FUNCTION "abvspu_AMP" : VOID
TITLE = Analoge Messwertverarbeitung
//
// Analoge Messwertverarbeitung
//
// History:
// --------
// 26-Aug-2005
// - Fehler bei cancel <out of range>
// 06-Nov-2004
// - Struktur DB180/181 erweitert (UndefGrp)
// 04-Feb-2004 (fixed)
// - TITLE = Messwert bilden (TYPE=1,...,15) - Eingangs-MS
//   U     DBX [AR1,P#21.7]; //unquittiert
//   // diese Abfrage entfernt! Relikt aus nicht optimierter SPU
//   U     #bUndefined;
//   SPB   M016;
//
// 16-Mai-2003 (added)
// - TITLE = Messwertänderung
//   Messwert-Kompensation
// - TITLE = Dyn. Limits
//   Refaktorisiert
//
// 05-Feb-2003 (redesign: Optimierung auf Geschwindigkeit)
//
AUTHOR : ab_rfe
FAMILY : AbvSpu
NAME : ANA_MS
VERSION : 3.2


VAR_INPUT
  OBJ : INT ;	// OBJ
  _TYPE : INT ;	// TYPE
  IN_VALUE : DWORD ;	// Analoger Eingangswert
  MSD_DBNO : WORD ;	// MS-Datenfeld (DB-Nummer)
  MSD_OFFSET : WORD ;	// MS-Datenfeld (Byteoffset)
  UNDEF_GRP : WORD ;	// Undefined Group
END_VAR
VAR_OUTPUT
  OUT_VALUE : WORD ;	// Ausgangswert (PAW)
  OUT_FLAG : BOOL ;	// Flag (new out_value)
END_VAR
VAR_TEMP
  help_db1 : WORD ;
  dwadr_db2_limits : WORD ;	// Anfang <Limits> in HilfsDB2
  r4NormVal : REAL ;	// aktueller Messwert (normiert)
  r4RawVal : REAL ;	// aktueller Messwert (Rohwert)
  bUndefined : BOOL ;
  bOutOfRange : BOOL ;
  bFadedOut : BOOL ;
  bAOValChanged : BOOL ;
  wRawVal : WORD ;	// Rohwert (gefiltert)
  wRawVal0 : WORD ;	// Rohwert (ungefiltert)
  dRawVal : DWORD ;
  yAnzStates : BYTE ;
  ySklRefNo : BYTE ;
  wParaDB : WORD ;	//DB-Nr. MS-Parameter
  dXmpStart : DWORD ;	// Zeiger auf Anfang MS-Datenfeld
  dXmpStates : DWORD ;	// Zeiger auf Zustandsdatenfeld
  dXmpAnaVars : DWORD ;	// Zeiger auf Zustandsdatenfeld
  dXmpLimits : DWORD ;	// Zeiger auf Zustandsdatenfeld
  dXmpLimitsEnd : DWORD ;	// Zeiger auf Zustandsdatenfeld
  dAR_UndefGrps : DWORD ;	// ptr -> Byte-Array UndefGrps
  dAR1 : DWORD ;
  dAR2 : DWORD ;
  wTmp : WORD ;
  wCycle1Ms : WORD ;
  bGA_Required : BOOL ;	// GA-Anforderung von DB104.DBX171.0
  yNewStatus : BYTE ;	//neuer Zustand
  yMB232 : BYTE ;
  yMB233 : BYTE ;
  r4LmtTemp : REAL ;
  r4LmtSaved : REAL ;
  r4LmtHysteresis : REAL ;
  wNewLvl : WORD ;
  wCurrDelay : WORD ;
  bValueAscending : BOOL ;	// Messwert steigend
  bValueDecreasing : BOOL ;	// Messwert fallend
  bLmtSaved : BOOL ;	// gerettetes Limit vorhanden
  bCheckOutOfRange : BOOL ;	// <OutOfRange> pruefen
  iObjKMS : INT ;	// Objektnummer Kompensations-MS
  r4ValKMS : REAL ;	// Messwert Kompensations-MS
  bRetValKMS : BOOL ;
  bLmtChanged : ARRAY  [1 .. 7 ] OF BOOL ;
  bLmtLast : BOOL ;
  wAnzLmts : INT ;
  r4MBA : REAL ;
  r4MBE : REAL ;
END_VAR
BEGIN
NETWORK
TITLE = Initialisierung

      L     "abvspu_DB_GLO".Cycle1Ms; // Zykluszeit (1ms-Aufl”sung)
      T     #wCycle1Ms;

      CLR   ;
      =     #bUndefined;

      L     #UNDEF_GRP;
      L     0;
      ==D   ;
      SPB   a001;

      L     "abvspu_DB_GLO".AR_UndefGrps;
      T     #dAR_UndefGrps;

      AUF   "abvspu_DB_GLO";
      LAR1  #dAR_UndefGrps;
      L     #UNDEF_GRP;
      +     -1;
      L     1; // 1 byte pro UndefGrp
      *D    ;
      SLD   3;
      +AR1  ;
      L     DBB [AR1,P#0.0];
      L     0;
      <>D   ;
      =     #bUndefined;

a001: NOP   0;
      L     #MSD_DBNO;
      T     #wParaDB;
      L     #MSD_OFFSET;
      SLD   3;
      T     #dXmpStart;
      LAR1  ;
      +AR1  P#26.0; //+13dw
      TAR1  #dXmpStates;

      CLR   ;
      =     #bOutOfRange;

      =     #bFadedOut;
      =     #bLmtSaved;

      =     #bValueAscending;
      =     #bValueDecreasing; // Nr. HilfsDB1 merken

      L     0; // HilfsDB1 aufrufen
      T     #yNewStatus; // Generalabfrage
      L     "spuDB_CFG".D_52; // DB195.DBW104
      T     #help_db1;

      AUF   DB [#help_db1];
      U     DBX  171.0;
      =     #bGA_Required;
NETWORK
TITLE = Feldbereiche berechnen

      AUF   DB [#wParaDB]; // Parameter-DB oeffnen
      LAR1  #dXmpStart;

      L     DBB [AR1,P#0.0]; // Kennung Ana-MS
      L     W#16#2; // Typ = ANA
      ==I   ;
      SPB   M001;
      L     W#16#B302; // falscher Feldtyp
      BEA   ;
M001: NOP   0;

      L     DBB [AR1,P#1.0]; // Anzahl Zustaende
      T     #yAnzStates;

      INC   1; // Zustand <OutOfRange>
      L     12; // 6DWs pro Zustand
      *I    ;
      SLD   3;
      L     #dXmpStates;
      +D    ;
      T     #dXmpAnaVars;
      L     34; //+17dw
      SLD   3;
      +D    ;
      T     #dXmpLimits;

      L     #yAnzStates;
      DEC   1;
      L     14; // Limitfeld (7dw)
      *I    ;
      SLD   3;
      L     #dXmpLimits;
      +D    ;
      T     #dXmpLimitsEnd; // ptr -> Ende Limitfeld

NETWORK
TITLE = Generalabfrage

      U     #bGA_Required; // Generalabfrage
      S     DBX [AR1,P#3.1]; // GA-Bit 'Zustand/Messwert'
      S     DBX [AR1,P#3.3]; // GA-Bit 'Nachparametrierung'
NETWORK
TITLE =Zeitverzögerung (current delay)

      UN    DBX [AR1,P#20.4]; // delay gestartet
      SPB   M002;
      L     DBW [AR1,P#22.0];
      L     #wCycle1Ms; // Zykluszeit (1ms-Auflösung)
      -I    ;
      T     DBW [AR1,P#22.0];
      L     0; // Stufe 1 abgearbeitet
      >I    ;
      SPB   M002;
      L     DBW [AR1,P#12.0]; // Zeitstufe 2
      +     -1;
      T     DBW [AR1,P#12.0];

      L     DBW [AR1,P#22.0];
      +     1000;
      T     DBW [AR1,P#22.0]; // Stufe 1 neu laden

M002: NOP   0;
NETWORK
TITLE = scancycle



NETWORK
TITLE =Grenzwerthysterese

      LAR2  #dXmpAnaVars; // ptr -> Analogvariablen
      L     DBD [AR2,P#8.0]; // Grenzwerthysterese/2
      T     #r4LmtHysteresis;

NETWORK
TITLE = Messwert bilden (TYPE=256) - Ausgangs-MS

      L     #_TYPE;
      L     256;
      <I    ;
      SPB   M003; // Eingangs-MS

      CLR   ;
      =     #OUT_FLAG;

      L     DBD [AR1,P#16.0]; // Messwert via SetValue()
      T     #r4NormVal;

      U     DBX [AR1,P#3.1]; // GA-Bit 'Zustand/Messwert'
      O(    ;
      L     #r4NormVal; // neuer Messwert
      L     DBD [AR1,P#4.0]; // aktueller Messwert
      <>R   ;
      )     ;
      =     #bAOValChanged;
      U     #bAOValChanged;
      SPB   M004;
      L     DBW [AR1,P#14.0];
      SPA   M005;
M004: NOP   0;
// Messwertaenderung=>Ausgang ansteuern;
// Messwert normieren (invers);
      L     1.000000e+000;
      L     DBD [AR2,P#0.0]; // a-Wert
      /R    ;
      L     #r4NormVal;
      *R    ;
      L     DBD [AR2,P#4.0]; // b-Wert
      +R    ;
      TRUNC ;
      T     #wRawVal;
      T     DBW [AR1,P#14.0];
      NOP   0;
//check range
M005: L     DBW [AR2,P#20.0]; //UNGR
      ITD   ;
      <D    ;
      SPB   M006;
      TAK   ;
      L     DBW [AR2,P#22.0]; //OBGR
      ITD   ;
      <=D   ;
      SPB   M007;
M006: NOP   0;
//OutOfRange
      L     16;
      T     #yNewStatus;
      SPA   M008;
M007: NOP   0;
// Rohwert ausgeben
      UN    #bAOValChanged;
      SPB   M008;
      CLR   ;
      L     #wRawVal;
      T     #OUT_VALUE;
      SET   ;
      =     #OUT_FLAG;
      SPA   M008;
NETWORK
TITLE = Messwert bilden (TYPE=1,...,15) - Eingangs-MS

M003: NOP   0;
      L     #_TYPE;
      L     15;
      >I    ; // wenn Type > 15 dann physikal.
      SPB   M009;

      NOP   0;
//Hardware-Signal einlesen;
      L     #IN_VALUE;
      T     #wRawVal;
      T     #wRawVal0;

      L     #_TYPE;
      SPL   M010;
      SPA   M011;
      SPA   M012; // HWM=1
      SPA   M011; // HWM=2 (PT100)
M010: NOP   0;
M011: NOP   0;
//Rohwert uebernehmen
      L     #wRawVal0;
      T     #wRawVal;
      SPA   M013;
M012: NOP   0;
//Rohwert maskieren
      L     #wRawVal0;
      UW    W#16#FFF8;
      T     #wRawVal;
      SPA   M013;
M013: NOP   0;
//bit 0,1,2 pruefen;
//bit 0: Ueberlauf;
//bit 1: Fehler
//bit 2: ?
//Undefined-Erkennung via UndefGrp
      U     #bUndefined;
      SPB   M014;
//Undefined-Erkennung via Rohwert
      L     #wRawVal0;
      L     W#16#7FFF;
      ==I   ;
      SPB   M014;
      TAK   ;
      L     W#16#8000;
      ==I   ;
      SPB   M014;
      SPA   M015;
M014: NOP   0;
      L     17; // undefiniert in UebergabeDW
      T     #yNewStatus;
M015: NOP   0;
      L     #wRawVal0;
      L     W#16#FFFE; // letztes Messwertbit ausblenden
      UW    ;
      T     #wRawVal; // aktueller Rohwert
      L     DBW [AR2,P#26.0]; // alter Rohwert
      ==I   ;
      =     DBX [AR1,P#20.2]; // Messwert gleich
      TAK   ;
      T     DBW [AR2,P#26.0]; // Messwert uebernehmen

      U     #bUndefined;
      SPB   M016;
      L     DBW [AR2,P#26.0]; // aktueller Messwert
      L     DBW [AR2,P#20.0]; // UNGR for out of range
      <I    ;
      SPB   M017;
      TAK   ;
      L     DBW [AR2,P#22.0]; // OBGR for out of range
      <=I   ;
      SPB   M016;
M017: NOP   0;
//OutOfRange
      L     16;
      T     #yNewStatus;
M016: NOP   0;
//normierten Messwert bilden;
      L     #wRawVal;
//konvertiere INT_16 nach INT_32;
//Wird Vorzeichen beruecksichtigt?
      ITD   ;
      T     #dRawVal;
//konvertiere INT_32 nach Real
      DTR   ;
      T     #r4RawVal;
      U     #bUndefined; // Messwert undefiniert
      SPB   M018;
      L     DBB [AR2,P#24.0]; // SKL-RefNo (wenn > 0 dann Normierung mit Polygon)
      T     #ySklRefNo;
      L     0;
      <>I   ;
      SPB   M019;
// Messwert normieren;
      L     DBD [AR2,P#0.0]; // a-Wert
      L     #r4RawVal; // x-Wert (Rohwert als Real)
      *R    ;
      L     DBD [AR2,P#4.0]; // b-Wert
      +R    ;
      T     #r4NormVal; // normierter Messwert
      SPA   M008; // ->Messwertvergleich
M019: NOP   0;
// normierter Messwert
      CALL "abvspu_XPO_NORM" (
           PODX                     := #ySklRefNo,
           ROHW                     := #r4RawVal,
           NRMV                     := #r4NormVal);

      SPA   M008;
M018: NOP   0;
      L     1.000000e+006;
      T     #r4NormVal; // normierter Messwert
      SPA   M008;
NETWORK
TITLE = Messwert bilden (physikalisch)

M009: NOP   0;
      L     #_TYPE;
      L     16; // physikal. Messwert 16 BIT
      ==I   ;
      SPB   M020;
// *** 32 BIT Wert ***;
      L     0.000000e+000;
      L     #IN_VALUE;
      +R    ;
      UN    UO; // Gleitpunktzahl gueltig
      SPB   REOK;
      L     #r4NormVal; // alten phys. Messwert beibehalten
REOK: T     #r4NormVal; // phys. Messwert (real)
      SPA   M021;
M020: NOP   0;
// *** 16 BIT Wert ***;
      L     #IN_VALUE;
      T     #wRawVal; // phys. Messwert (int16)
      ITD   ;
      T     #dRawVal;
      DTR   ; // ->real
      T     #r4NormVal; // Wert als Real
//*** Start: OutOfRange (pysikalisch) ***//
M021: NOP   0;

      L     DBB [AR2,P#24.0]; // SKL-RefNo (wenn > 0 dann Normierung mit Polygon)
      T     #ySklRefNo;
      L     0;
      ==I   ;
      SPB   M022;
// normierter Messwert
      CALL "abvspu_XPO_NORM" (
           PODX                     := #ySklRefNo,
           ROHW                     := #r4NormVal,
           NRMV                     := #r4NormVal);

      AUF   DB [#wParaDB];
      LAR1  #dXmpStart;
      LAR2  #dXmpAnaVars;

M022: NOP   0;
      L     #r4NormVal;
      L     DBD [AR2,P#0.0]; //Messbereichsanfang
      <R    ;
      SPB   M023;
      TAK   ;
      L     DBD [AR2,P#4.0]; //Messbereichsende
      <=R   ;
      SPB   M024;
M023: NOP   0;
//OutOfRange
      L     16;
      T     #yNewStatus;
      SPA   M027;
M024: NOP   0;
      UN    #bUndefined;
      SPB   M027;
      L     17; // undefiniert in UebergabeDW
      T     #yNewStatus;
M027: NOP   0;
//*** Ende : OutOfRange (pysikalisch) ***//
NETWORK
TITLE = Messwertaenderung?

M008: NOP   0;

      LAR2  #dXmpAnaVars;
      L     DBW [AR2,P#28.0]; // ObjNo Kompensations-MS
      L     0;
      ==I   ;
      SPB   wei3;
//
// Kompensations-MS
      TAK   ;
      T     #iObjKMS;

      CALL "GetValueR_ex" (
           obj                      := #iObjKMS,
           rVal                     := #r4ValKMS,
           bOk                      := #bRetValKMS);

      UN    #bRetValKMS;
      SPB   wei3;

// cancel <out of range>
//    L     0;
//    T     #yNewStatus;

      L     #r4NormVal;
      L     #r4ValKMS;
      +R    ;
      T     #r4NormVal;
      SPA   wei3;

// raw value zurückrechnen, um 'out of range' zu prüfen
      L     1.000000e+000;
      L     DBD [AR2,P#0.0]; // a-Wert
      /R    ;
      L     #r4NormVal;
      *R    ;
      L     DBD [AR2,P#4.0]; // b-Wert
      +R    ;
      TRUNC ; // raw value

//check range
      L     DBW [AR2,P#20.0]; //UNGR
      ITD   ;
      <D    ;
      SPB   k001;
      TAK   ;
      L     DBW [AR2,P#22.0]; //OBGR
      ITD   ;
      <=D   ;
      SPB   wei3;
k001: NOP   0;
//OutOfRange
      L     16;
      T     #yNewStatus;

wei3: NOP   0;
      UN    DBX [AR1,P#3.2]; // Simulationsmodus?
      SPB   M025;
      L     #OBJ; // ObjNo
      T     #wTmp;
      L     #r4NormVal; // Akt. Messwert -> Akku1
      CALL "abvspu_AMPSIM" (
           OBJ                      := #wTmp);

      T     #r4NormVal; // Aktueller Messwert
M025: NOP   0;
      L     #r4NormVal;
      L     DBD [AR1,P#4.0]; //alter Messwert
      ==R   ;
      =     DBX [AR1,P#20.2]; // Messwert gleich

// force value changed, if <status==0> or <GA-Bit>
      L     DBW [AR1,P#8.0];
      L     0;
      ==I   ;
      O     DBX [AR1,P#3.1];
      O     DBX [AR1,P#3.4]; // force value change
      R     DBX [AR1,P#20.2]; // Messwert gleich

      UN    DBX [AR1,P#20.2];
      =     DBX [AR1,P#20.7]; // Messwert eintragen

      U     DBX [AR1,P#3.4];
      R     DBX [AR1,P#3.4];
NETWORK
TITLE = Dynamische Limits

      L     0;
      L     DBB [AR2,P#33.0];
      ==I   ; // dynamische Limits vorhanden?
      SPB   M026;

      CLR   ;
      =     #bLmtChanged[1];
      =     #bLmtChanged[2];
      =     #bLmtChanged[3];
      =     #bLmtChanged[4];
      =     #bLmtChanged[5];
      =     #bLmtChanged[6];
      =     #bLmtChanged[7];

//Messbereichsanfang, -ende ermitteln
      L     #_TYPE;
      L     16;
      >=I   ;
      O(    ;
      L     #ySklRefNo; // Skaliergruppe
      L     0;
      >I    ;
      )     ;
      SPB   RNG2;
//Messbereich aus Gradient/Offset ermitteln;
//MBA=offset+(gradient*UNGR)
//MBE=(gradient*OBGR)+offset
      L     DBW [AR2,P#20.0]; //UNGR
      ITD   ;
      DTR   ;
      L     DBD [AR2,P#0.0]; //Gradient
      *R    ;
      L     DBD [AR2,P#4.0]; //Offset
      +R    ;
      T     #r4MBA;
//
      L     DBW [AR2,P#22.0]; //OBGR
      ITD   ;
      DTR   ;
      L     DBD [AR2,P#0.0]; //Gradient
      *R    ;
      L     DBD [AR2,P#4.0]; //Offset
      +R    ;
      T     #r4MBE;
      SPA   RNGX;
RNG2: NOP   0;
      L     DBD [AR2,P#0.0];
      T     #r4MBA;
      L     DBD [AR2,P#4.0];
      T     #r4MBE;

RNGX: NOP   0;

      L     #yAnzStates; // Anzahl Zustaende
      +     -1; // Anzahl Limits
      T     #wAnzLmts;

      UN    DBX [AR2,P#33.1]; // 1. Limit dynamisch
      SPB   LIM2;


      CALL "abvspu_DYLI" (
           IN_Obj                   := #OBJ,
           IN_wParaDB               := #wParaDB,
           IN_dXmpAnaVars           := #dXmpAnaVars,
           IN_dXmpLimits            := #dXmpLimits,
           IN_RngStrt               := #r4MBA,
           IN_RngEnd                := #r4MBE,
           IN_wLmtNo                := 1,
           IN_wAnzLmts              := #wAnzLmts,
           OUT_bLmtChanged          := #bLmtChanged[1],
           OUT_bLmtLast             := #bLmtLast);


      U     #bLmtLast;
      SPB   M026;

LIM2: UN    DBX [AR2,P#33.2]; // 2. Limit dynamisch
      SPB   LIM3;

      CALL "abvspu_DYLI" (
           IN_Obj                   := #OBJ,
           IN_wParaDB               := #wParaDB,
           IN_dXmpAnaVars           := #dXmpAnaVars,
           IN_dXmpLimits            := #dXmpLimits,
           IN_RngStrt               := #r4MBA,
           IN_RngEnd                := #r4MBE,
           IN_wLmtNo                := 2,
           IN_wAnzLmts              := #wAnzLmts,
           OUT_bLmtChanged          := #bLmtChanged[2],
           OUT_bLmtLast             := #bLmtLast);

      U     #bLmtLast;
      SPB   M026;

LIM3: UN    DBX [AR2,P#33.3]; // 3. Limit dynamisch
      SPB   LIM4;

      CALL "abvspu_DYLI" (
           IN_Obj                   := #OBJ,
           IN_wParaDB               := #wParaDB,
           IN_dXmpAnaVars           := #dXmpAnaVars,
           IN_dXmpLimits            := #dXmpLimits,
           IN_RngStrt               := #r4MBA,
           IN_RngEnd                := #r4MBE,
           IN_wLmtNo                := 3,
           IN_wAnzLmts              := #wAnzLmts,
           OUT_bLmtChanged          := #bLmtChanged[3],
           OUT_bLmtLast             := #bLmtLast);

      U     #bLmtLast;
      SPB   M026;

LIM4: UN    DBX [AR2,P#33.4]; // 4. Limit dynamisch
      SPB   LIM5;

      CALL "abvspu_DYLI" (
           IN_Obj                   := #OBJ,
           IN_wParaDB               := #wParaDB,
           IN_dXmpAnaVars           := #dXmpAnaVars,
           IN_dXmpLimits            := #dXmpLimits,
           IN_RngStrt               := #r4MBA,
           IN_RngEnd                := #r4MBE,
           IN_wLmtNo                := 4,
           IN_wAnzLmts              := #wAnzLmts,
           OUT_bLmtChanged          := #bLmtChanged[4],
           OUT_bLmtLast             := #bLmtLast);

      U     #bLmtLast;
      SPB   M026;
      SPA   LIM5;

M026: SPA   M031;
LIM5: UN    DBX [AR2,P#33.5]; // 5. Limit dynamisch
      SPB   LIM6;

      CALL "abvspu_DYLI" (
           IN_Obj                   := #OBJ,
           IN_wParaDB               := #wParaDB,
           IN_dXmpAnaVars           := #dXmpAnaVars,
           IN_dXmpLimits            := #dXmpLimits,
           IN_RngStrt               := #r4MBA,
           IN_RngEnd                := #r4MBE,
           IN_wLmtNo                := 5,
           IN_wAnzLmts              := #wAnzLmts,
           OUT_bLmtChanged          := #bLmtChanged[5],
           OUT_bLmtLast             := #bLmtLast);

      U     #bLmtLast;
      SPB   M031;
LIM6: UN    DBX [AR2,P#33.6]; // 6. Limit dynamisch
      SPB   LIM7;

      CALL "abvspu_DYLI" (
           IN_Obj                   := #OBJ,
           IN_wParaDB               := #wParaDB,
           IN_dXmpAnaVars           := #dXmpAnaVars,
           IN_dXmpLimits            := #dXmpLimits,
           IN_RngStrt               := #r4MBA,
           IN_RngEnd                := #r4MBE,
           IN_wLmtNo                := 6,
           IN_wAnzLmts              := #wAnzLmts,
           OUT_bLmtChanged          := #bLmtChanged[6],
           OUT_bLmtLast             := #bLmtLast);

      U     #bLmtLast;
      SPB   M031;
LIM7: UN    DBX [AR2,P#33.7]; // 7. Limit dynamisch
      SPB   M031;

      CALL "abvspu_DYLI" (
           IN_Obj                   := #OBJ,
           IN_wParaDB               := #wParaDB,
           IN_dXmpAnaVars           := #dXmpAnaVars,
           IN_dXmpLimits            := #dXmpLimits,
           IN_RngStrt               := #r4MBA,
           IN_RngEnd                := #r4MBE,
           IN_wLmtNo                := 7,
           IN_wAnzLmts              := #wAnzLmts,
           OUT_bLmtChanged          := #bLmtChanged[7],
           OUT_bLmtLast             := #bLmtLast);

M031: NOP   0;

      O     #bLmtChanged[1];
      O     #bLmtChanged[2];
      O     #bLmtChanged[3];
      O     #bLmtChanged[4];
      O     #bLmtChanged[5];
      O     #bLmtChanged[6];
      O     #bLmtChanged[7];
      S     DBX [AR1,P#20.1]; // Grenzwertänderung anzeigen

NETWORK
TITLE = Ein-/Ausblenden (fade in/out)

      UN    DBX [AR1,P#3.0]; // 1=aus, 0=eingeblendet
      SPB   M034; //eingeblendet
      SET   ;
      =     #bFadedOut;
      L     18; // Status <ausgeblendet>
      T     #yNewStatus;
//NEXT:
M034: NOP   0;
NETWORK
TITLE = Limit allgemein

      U     #bFadedOut; // ausgeblendet
      SPB   M035; // Sendehysterese Messwert bearbeiten
      O(    ;
      L     #yAnzStates; //Anzahl Zustaende
      L     1;
      <=I   ;
      )     ;
      O(    ;
      L     #yNewStatus;
      L     W#16#1F;
      UW    ; // wenn kein
      L     8; // normaler Zustaend
      >=I   ; // dann keine Limitbearbeitung
      )     ;
      =     #bCheckOutOfRange; // out of range pruefen
      SPB   M035;
      U     DBX [AR1,P#9.4]; // Bit 1&4 gesetzt = 18 (ausgeblendet)
      U     DBX [AR1,P#9.1];
      UN    DBX [AR1,P#3.0]; // Kommando: einblenden
      SPB   M036;
      U     DBX [AR1,P#20.1]; // Limit geaendert
      SPB   M036;
      UN    DBX [AR1,P#20.2]; // Messwert gleich
      SPB   M035;
      L     DBW [AR1,P#20.0]; // letzter bearbeiteter Zustand
      T     #yNewStatus;
      SPA   M037;

M035: NOP   0;
      L     #r4NormVal; // aktueller Messwert
//    L     DBD    4; // gemeldeter Messwert
      L     DBD [AR2,P#16.0]; // gesendeter Messwert
      >R    ;
      =     #bValueAscending; // Messwert steigend

      U     #bValueAscending;
      SPB   M038;
      TAK   ;
M038: NOP   0;
      -R    ;
//???????      T     DBD  172                    // positive Messwertaenderung
      L     DBD [AR2,P#12.0]; // Sendehysterese
      <R    ;
      R     DBX [AR1,P#20.7]; // Messwert eintragen
      U     #bFadedOut; // ausgeblendet
      O     #bCheckOutOfRange; //1 Zustand
      R     #bValueAscending; // Messwert steigend
      SPB   M039; //ENDE (keine Zustandsbearbeitung)
M036: NOP   0;
      U     DBX [AR1,P#20.4]; // Zeit laeuft ...
      SPB   M040;
//alter (gemeldeter) Zustand;
      L     DBW [AR1,P#8.0];
      SPA   M041;
M040: NOP   0;
//neuer Zustand (Verz.Zeit laeuft);
      L     DBB [AR1,P#21.0];
M041: NOP   0;
      L     W#16#1F;
      UW    ;
      T     #yMB232; // Zustand ohne BIT 5-15
      U     DBX [AR1,P#20.1]; // dyn. Limit geaendert
      SPB   M042;
      L     16; // out of range?
      <I    ;
      SPB   M043;
//WEI2:
M042: NOP   0;
      UN    #bValueAscending; // Messwert steigend
      S     #bValueAscending;
M044: NOP   0;

      TAR1  #dAR1;
      LAR1  #dXmpStates;

      L     #yAnzStates; // Anzahl Zustaende
      DEC   1;
      L     12; // Laenge Zustandsfeld (6dw)
      *I    ;
      SLD   3;
      +AR1  ; // ptr -> letztes Zustandsdatenfeld

      L     DBB [AR1,P#4.0]; // Alarmlevel
      T     #yMB233; // eingetragener Alarmlevel

      LAR1  #dAR1; // ptr -> Allgemeine MS-Daten

      O     #bValueAscending; // steigend forcieren
      ON    #bValueAscending;
      =     #bValueAscending;
      SPB   M045;
      L     #yAnzStates; // Anzahl Zustaende
      +     1; // + out of range
      T     #yMB232; // Zustandspos. fuer out of range
      SPA   M046;
M045: NOP   0;
      L     #yAnzStates; // Anzahl Zustaende
      T     #yMB232;
      SPA   M046;
M043: NOP   0;
      TAK   ; // wenn eingetragener Zustand
      L     0; // gleich 0 dann Berechnung ueber
      ==I   ; // Anzahl der Zustaende
      SPB   M044;

      TAR1  #dAR1;
      LAR1  #dXmpStates;

      L     #yMB232; // eingetragener Zustand
      +     -1; // -1
      L     12; // Laenge Statefeld (6dw)
      *I    ;
      SLD   3;
      +AR1  ; // ptr -> Zustandsdatenfeld
      L     DBB [AR1,P#4.0]; // Alarmlevel
      T     #yMB233; // eingtragener Alarmlevel

      LAR1  #dAR1; // ptr -> Allgemeine MS-Daten

      L     #yMB232;
      L     16;
      <I    ; // normaler Zustand
      SPB   M046;

      L     1; // Zustand fuer Bearbeitung auf
      T     #yMB232; // 1 setzen

      O     #bValueAscending; // Durchsuchungsrichtung auf
      ON    #bValueAscending;
      =     #bValueAscending; // steigend stellen

      L     0; // Alarmlevel fuer Bearbeitung
      T     #yMB233; // auf 0 setzen

M046: NOP   0;
      U     DBX [AR1,P#20.1]; // Limit geaendert
      R     DBX [AR1,P#20.1];
      UN    #bValueAscending; // Durchsuchungsrichtung steigend
      =     #bValueDecreasing; // Bearbeitung fallend
      SPA   M039; //ENDE;

M037: NOP   0;
      T     #yNewStatus;

M039: NOP   0;
NETWORK
TITLE = Limit steigend

      UN    #bValueAscending; // Messwert steigend
      SPB   M047;
      L     1; // kleinster Zustand erreicht
      L     #yMB232; // gemeldeter Zustand
      >=I   ;
      SPB   M048;
// ** Berechnung der Limitposition (Zustand>1)

      TAR2  #dAR2;
      LAR2  #dXmpLimits; // ptr -> Limitfeld

      +     -2; // Z2/L1, Z3/L2, ..., Z8/L7
      L     14; // Laenge Limitfeld (7dw)
      *I    ;
      SLD   3;
      +AR2  ; // ptr -> Limitfeld

M049: NOP   0;
      L     DBD [AR2,P#0.0]; // Limit auslesen
      T     #r4LmtTemp;
      L     #r4LmtHysteresis; // Hysterese/2
      +R    ;
      L     #r4NormVal; // Messwert
      >R    ;
      SPB   M048;

      L     #yMB232;
      DEC   1;
      T     #yMB232;

      L     -112; // ein Feld (7dw) zurueck (7*2*8)
      +AR2  ;
      TAR2  ;
      L     #dXmpLimits; // ptr -> Limitfeld (Anfang)
      <D    ;
      SPB   M048;
      SPA   M049; // LOOP
M048: NOP   0;
      L     #yMB232;
      +     -1; // -1
      L     12; // Laenge Statefeld (6dw)
      *I    ;
      SLD   3;
      TAR1  #dAR1;
      LAR1  #dXmpStates;
      +AR1  ; // prt -> Statusfeld
      L     DBW [AR1,P#0.0]; // neue Delays
      T     #wCurrDelay;

      L     DBW [AR1,P#4.0]; // neuer Alarmlevel
      T     #wNewLvl;

      L     #yMB232; // aktueller Zustand
      T     #yNewStatus;

      LAR2  #dAR2;
      LAR1  #dAR1;

M047: NOP   0;
NETWORK
TITLE = Limit fallend

      UN    #bValueDecreasing; // Bearbeitung fallend
      SPB   M050;
      L     #yAnzStates; // Anzahl Zustaende
      L     #yMB232; // aktueller Zustand
      <=I   ;
      SPB   M051;

      TAR2  #dAR2;
      LAR2  #dXmpLimits; // ptr -> Limitfeld

      +     -1; // -1
      L     14; // Laenge Limitfeld (7dw)
      *I    ;
      SLD   3;
      +AR2  ; // ptr -> Limitfeld

//LOOP:
M052: NOP   0;
      L     DBD [AR2,P#0.0]; // Limit auslesen
      T     #r4LmtTemp;
      L     #r4LmtHysteresis; // Hysterese/2
      -R    ;
      L     #r4NormVal; // Messwert
      <R    ;
      SPB   M051;

      L     #yMB232; // Zustand
      INC   1; // -1
      T     #yMB232;

      +AR2  P#14.0; // +7DWs
      TAR2  ;
      L     #dXmpLimitsEnd; // ptr -> Ende Limitfeld
      >=D   ;
      SPB   M051;
      L     #r4LmtTemp; // ermitteltes Limit retten
      T     #r4LmtSaved;
      UN    #bLmtSaved;
      S     #bLmtSaved; // gerettetes Limit vorhanden
      SPA   M052; // LOOP

M051: NOP   0;
      UN    #bLmtSaved;
      SPB   M053;
      L     #r4LmtSaved; // gerettetes Limit
      T     #r4LmtTemp; // zurueckschreiben

M053: NOP   0;
      L     #yMB232;
      +     -1; // -1
      L     12; // Laenge Statefeld (6dw)
      *I    ;
      SLD   3;
      TAR1  #dAR1;
      LAR1  #dXmpStates;
      +AR1  ; // prt -> Statusfeld

      L     DBW [AR1,P#0.0]; // neue Delays
      T     #wCurrDelay; // neue Delays
      L     DBW [AR1,P#4.0]; // neuer Alarmlevel
      T     #wNewLvl;

      L     #yMB232; // aktueller Zustand
      T     #yNewStatus;

      LAR2  #dAR2;
      LAR1  #dAR1;

M050: NOP   0;
NETWORK
TITLE = Limit out of range

      UN    #bCheckOutOfRange; // out of range pruefen
      SPB   M054;
      L     #yNewStatus; // aktueller Zustand
      L     W#16#1F;
      UW    ;
      L     0;
      <>I   ;
      SPB   M055;
//Aktueller Zustand=0 (Anzahl Zustaende=1);
      L     1;
      T     #yNewStatus;
      L     0;
      T     #wNewLvl;
      T     #wCurrDelay;
      SPA   M054;
M055: NOP   0;
      TAK   ;
      L     16; // outofrange
      ==I   ;
      SPB   M056;
      TAK   ;
      L     17; // undefiniert
      <>I   ;
      SPB   M054;
// dwadr HilfsDB2 <Limits> = Endadresse States HDB2
M056: NOP   0;
      LAR2  #dXmpAnaVars;
      L     -64; // -4dw (4x2x8)
      +AR2  ; // ptr -> alarmlevel
      L     DBW [AR2,P#0.0]; // Alarmlevel
      T     #wNewLvl;
      L     -32; // 2DWs zurueck (2x2x8)
      +AR2  ;
      L     DBW [AR2,P#0.0]; // Delays
      T     #wCurrDelay;

M054: NOP   0;
NETWORK
TITLE = Aufruf Basisfunktion (Zustands-/Grenzwertbehandlung)

      AUF   DB [#wParaDB];
      LAR2  #dXmpStart; //Zeiger auf MS-Parameter

      CALL "abvspu_STALIM" (
           IN_Obj                   := #OBJ,
           IN_NewState              := #yNewStatus,
           IN_NewValue              := #r4NormVal,
           IN_NewLvl                := #wNewLvl,
           IN_CurrentDly            := #wCurrDelay);
END_FUNCTION

FUNCTION "abvspu_UDP_RECV" : BOOL
TITLE = UDP_RECV
//
// Funktion:
// - UDP-Receive
//
// Historie
// # 23-Jan_2006 (added)
// - abvspu_UDP_SendRecvDT: Empfangen von Uhrzeit-Synchronisations-Telegrammen
// # 22-Apr-2004 (added)
// - AGxRECV <Fallunterscheidung CPU 300/400>
//
AUTHOR : ab_rfe
FAMILY : AbvSpu
NAME : UDP_RECV
VERSION : 2.1


VAR_TEMP
  wDbtNo : WORD ;
  wI : WORD ;
  wAnzPC : WORD ;	// Anzahl PCs
  wPcMax : WORD ;	// Maximale Anzahl PCs
  wSrcDb : WORD ;	// Quell_DB
  wDstDb : WORD ;	// Ziel_DB
  wSrcOffs : WORD ;	// DW-Nr. Quell_DB
  wDstOffs : WORD ;	// DW-Nr. Ziel_DB
  wAnzWords : WORD ;	// Anzahl DWs (CopyDB)
  wAnzBytes : WORD ;	// Anzahl Bytes (CopyDB)
  bWdogTime : BOOL ;
  bClrAendDBs : BOOL ;	//AendDBs leeren
  recv_error : BOOL ;
  recv_ndr : BOOL ;
  recv_status : WORD ;
  recv_len : INT ;
  dwTmp : DWORD ;
  wRcvDB : WORD ;
  wRcvDBLen : WORD ;
  wRecvDataLenB : WORD ;
  wDbNo_UDP_Control : WORD ;
  wPcStationNumber : WORD ;	//Stationsnummer Visu-PCs: 1..32
  bNotForMe : BOOL ;	//Telegramm muss ignoriert, aber Zähler erhöht werden
  wReturnMark : WORD ;
  wTmp : WORD ;
  wDBNo : WORD ;
END_VAR
BEGIN
NETWORK
TITLE = Initialisierung

      U     DB195.DBX  186.0; // UDP-Initialisierung okay?
      BEB   ;

//***********
//uHo
      CLR   ;
      =     #RET_VAL; // Clear return value 'New Data Received'
//***********

      CALL "abvspu_UDP_SendRecvDT" (// TimeSyncTele empfangen
           bSend                    := FALSE);

      L     "spuDB_CFG".D_90; // DB195.DBW180 (DB-SAPI/UDP)
      T     #wDbNo_UDP_Control;

//S7-Wdog-Zaehler;
      L     "abvspu_DB_UDP".S7_WDOG;
      INC   1;
      T     "abvspu_DB_UDP".S7_WDOG;
// Anzahl PCs;
      L     "spuDB_CFG".D_81; // DB195.DBW 162
      T     #wAnzPC;
      CLR   ;
      =     #bWdogTime;
//PC online?;
      L     "abvspu_DB_GLO".Cycle1Ms; // Zeit des letzten Zyklus in Anzahl ms
      L     "abvspu_DB_UDP".WDOG_TIME;
      +D    ;
      T     "abvspu_DB_UDP".WDOG_TIME;
      L     5000; // 5sec
      <D    ;
      SPB   a000;
//Zeit abgelaufen;
//WDOG_PC* pruefen;
//;
      SET   ;
      =     #bWdogTime;
//;
a000: NOP   0;
      L     "spuDB_CFG".D_90; // DB195.DBW 180
      T     #wDbtNo; // DB-Nr. UDP-Datenbaustein
      L     32;
      T     #wPcMax;
      L     0;
      T     #wI;
//DB-Nr. Ziel-DB (Receive)
      L     "spuDB_CFG".D_55; // DB195.DBW 110 = Recv_DB
      T     #wDstDb;
      L     0;
      T     #wDstOffs;

NETWORK
TITLE =Receive

      UN    "abvspu_DB_UDP".bDoRecvTele; // Test-Flag
      SPB   rcv1; // UDP-Receive
// Simulation UDP-Empfangsdaten
      CLR   ;
      =     "abvspu_DB_UDP".bDoRecvTele;

      LAR2  "abvspu_DB_UDP".dPtrRecvTele1;

      L     "abvspu_DB_UDP".dwTest_SenderId;
      T     D [AR2,P#0.0];

      L     "abvspu_DB_UDP".dwTest_PacketId;
      T     D [AR2,P#4.0];

      L     "abvspu_DB_UDP".dwTest_ReceiverId;
      T     D [AR2,P#8.0];

      L     "abvspu_DB_UDP".dwTest_PacketType;
      T     D [AR2,P#12.0];

      L     "abvspu_DB_UDP".dwTest_TotalPacketLength;
      T     D [AR2,P#16.0];

      L     "abvspu_DB_UDP".dwTest_PartialPacketId;
      T     D [AR2,P#20.0];

      L     "abvspu_DB_UDP".dwTest_NettoDataLen;
      T     #dwTmp;

      LAR1  "abvspu_DB_UDP".dPtrTest_NettoData;
      +AR2  P#24.0;

lp1:  L     0;
      L     #dwTmp;
      ==I   ;
      SPB   rcv2;
      +     -1;
      T     #dwTmp;
      L     DBB [AR1,P#0.0];
      T     DBB [AR2,P#0.0];
      +AR2  P#1.0;
      +AR1  P#1.0;
      SPA   lp1;

// immer auf der ersten UDP-Verbindung empfangen (Port local/remote!)

rcv1: CALL "abvspu_AGxRECV" (
           ID                       := "abvspu_DB_UDP".wFirstConnection,
           LADDR                    := "abvspu_DB_UDP".wLAddr[1],
           RECV                     := "abvspu_DB_UDP".RecvTele[1],
           NDR                      := #recv_ndr,
           ERROR                    := #recv_error,
           STATUS                   := #recv_status,
           LEN                      := #recv_len);

      UN    #recv_ndr;
      O     #recv_error;
      SPB   WDOG; // nichts oder mit Fehler empfangen

//***********
//uHo
      SET   ;
      =     #RET_VAL; // Set Return value 'New Data Received'
//***********

// Check Receiver-ID (must be in range 1...64)
rcv2: NOP   0;

      CLR   ;
      =     #bNotForMe;

      L     "abvspu_DB_UDP".RecvTele[1].TeleHeader.ReceiverId;
      TAD   ;
      L     "spuDB_CFG".D_54; // station number of S7 (DB195.DBW 108)
      <>D   ;
      U(    ;
      TAK   ;
      L     L#-1; // broadcast
      <>D   ;
      )     ;

      S     #bNotForMe;

// Check Sender-ID (must be in range 101...132)
      L     "abvspu_DB_UDP".RecvTele[1].TeleHeader.SenderId;
      TAD   ;
      L     100;
      <=D   ;
      O(    ;
      TAK   ;
      L     133;
      >=D   ;
      )     ;
      SPB   WDOG;

      L     "abvspu_DB_UDP".RecvTele[1].TeleHeader.SenderId;
      TAD   ;
      L     100;
      -D    ;
      T     #wPcStationNumber; // range is 1..32 (Sender-ID - 100)

// Check telegram length <-> TotalPacketLength
      L     #recv_len;
      L     24;
      -D    ;
      L     "abvspu_DB_UDP".RecvTele[1].TeleHeader.TotalPacketLength;
      TAD   ;
      <>D   ;
      SPB   WDOG;

// check packet type
      L     "abvspu_DB_UDP".RecvTele[1].TeleHeader.PacketType;
      TAD   ;
      SPL   spxx;
      SPA   ntto; //0=netto data
      SPA   rb; //1=rollback-request
      SPA   ls; //2=life sign
      SPA   tolo; //3=packet id too low
spxx: SPA   WDOG; //unknown type

// Rollback-Request (PacketID ist egal)
rb:   NOP   0;

      U     #bNotForMe;
      SPB   WDOG;

      L     "abvspu_DB_UDP".wRollbackRequestsFromPC;
      L     1;
      +D    ;
      T     "abvspu_DB_UDP".wRollbackRequestsFromPC;

      SET   ;
      =     "abvspu_DB_UDP".bRecvRollbackRequest; // is handled in FC192

// Rollback-PacketID steht in Nettodaten abData[0..3]
      LAR1  "abvspu_DB_UDP".dPtrRecvTele1;
      L     D [AR1,P#24.0];
      T     "abvspu_DB_UDP".dwRollbackPacketId; // Rollback-PacketID

      SPA   WDOG;

// Life sign
// OS1: SenderID=101
ls:   NOP   0;

      U     #bNotForMe;
      SPB   WDOG;

      L     0; // return to r000 !
      T     #wReturnMark;
      SPA   rrrr;
r000: NOP   0; // return to here

WDOG: NOP   0;
// no receive or error
      UN    #bWdogTime;
      BEB   ;
// Wdog time expired, handle pc- online status
      L     "abvspu_DB_UDP".PC_RecvTeleFlag;
      L     "abvspu_DB_UDP".PC_ONLINE;
      UD    ;
      T     "abvspu_DB_UDP".PC_ONLINE;

      L     0;
      T     "abvspu_DB_UDP".PC_RecvTeleFlag;

      L     0;
      T     "abvspu_DB_UDP".WDOG_TIME;

      BEA   ;

NETWORK
TITLE =packet type <netto data>

ntto: NOP   0; // packet type <netto data>
// alle Telegramme mithören und LastRecvPacketId erhöhen
// auch wenn Telegramm für eine andere Station ist.
// Erst später U #bNotForMe abfragen!


      L     1; // return to r001 !
      T     #wReturnMark;
      SPA   rrrr;
r001: NOP   0; // return to here


      L     6;
      L     "abvspu_DB_UDP".RecvTele[1].TeleHeader.TotalPacketLength;
      TAD   ;
      <>D   ;
      SPB   n001; // keine GA

      L     DB190.DBB 1585; // Inhalt von Netto-Byte 1
      L     W#16#11; // Kennung für GA
      <>D   ;
      SPB   n001; // keine GA

// jetzt LastRecvDataPacketId auf -1 setzen:
// GA muss unabhängig von PacketId bearbeitet werden.

      TAR1  #dwTmp;
      L     #wPcStationNumber;
      L     1;
      -D    ;
      L     32;
      *D    ;
      L     "abvspu_DB_UDP".dPtrLastRecvDataPacketId; // Zeiger auf PC-PacketId-Variablen im DB190
      +D    ;
      LAR1  ;

      AUF   "abvspu_DB_UDP";
      L     L#-1;
      T     DBD [AR1,P#0.0];

      LAR1  #dwTmp;

// und (GA-Request-)Telegramm als initielles bearbeiten

n001: NOP   0;
      L     #wPcStationNumber;
      L     1;
      -D    ;

      L     P#4.0;
      *D    ;

      L     "abvspu_DB_UDP".dPtrLastRecvDataPacketId; // Zeiger auf PC-PacketId-Variablen im DB190
      +D    ;
      LAR1  ;

      L     "abvspu_DB_UDP".RecvTele[1].TeleHeader.PacketId;
      L     L#-1;
      ==D   ; // accept first tele
      SPB   ok;

      TAK   ;
      L     0;
      ==D   ;
      SPB   ok; // first tele from Udp2Av has packet id 0 !


      AUF   "abvspu_DB_UDP";
      L     DBD [AR1,P#0.0];

      T     #dwTmp; // == last received data packet id
      L     L#-1;
      ==D   ; // first tele -> accept any value for packet-id
      SPB   ok;

      TAK   ;
      L     "abvspu_DB_UDP".RecvTele[1].TeleHeader.PacketId;
      TAD   ;
      TAK   ; // Akku1 == neu, Akku2 == alt
      -D    ; // Akku1 == neu - alt

      L     L#1;
      ==D   ; // neu - alt = 1
      SPB   ok;

      TAK   ;
      L     L#-10;
      <=D   ; // neu - alt <= -10  <->  neu <= alt - 10
      SPB   ok; // neu = ..., alt-13, alt-12, alt-11 (adaptiere PacketId)

      TAK   ;
      L     1;
      <D    ; // neu - alt < 1  <->  neu < alt + 1
      SPB   ign; // neu = alt-9, alt-8, alt-7, ..., alt-1, alt

// jetzt: neu = alt+2, alt+3, alt+3, ...
      SET   ;
      =     "abvspu_DB_UDP".bSendRollbackRequest;
      L     #dwTmp;
      +     1;
      T     "abvspu_DB_UDP".dwRollbackReqPacketId;


      L     "abvspu_DB_UDP".RecvTele[1].TeleHeader.SenderId;
      TAD   ;
      T     "abvspu_DB_UDP".dwRollbackReqReceiverId;

      SPA   ign;

// UDP-Nettodaten in Recv-DB (DB135) umspeichern
ok:   NOP   0;

      L     "abvspu_DB_UDP".RecvTele[1].TeleHeader.PacketId;
      TAD   ;
      T     DBD [AR1,P#0.0];
      U     #bNotForMe;
      SPB   WDOG;

      L     "spuDB_CFG".D_55; // DB195.DBW110 = RecvDB-No
      T     #wRcvDB;

      AUF   DI [#wRcvDB]; // Destination
      L     DILG;
      T     #wRcvDBLen;

      L     #wRcvDBLen;
      L     "abvspu_DB_UDP".RecvTele[1].TeleHeader.TotalPacketLength;
      TAD   ;
      T     #wRecvDataLenB; // Anzahl Bytes Nettodaten
      <D    ;
      SPB   ign; // Recv-DB too small

      NOP   0;


// *** strcpy *************************************************

      LAR1  "abvspu_DB_UDP".dPtrRecvTele1; // Ptr-Source (hallo: bei Redundanz?!?)
      +AR1  P#24.0; // UDP-Header überspringen
      LAR2  P#0.0; // Ptr-Destination

      AUF   DB [#wDbNo_UDP_Control]; // Source
      AUF   DI [#wRcvDB]; // Destination

      L     #wRecvDataLenB;
      T     #dwTmp; // Anzahl Bytes
SCPY: L     0;
      L     #dwTmp;
      ==I   ;
      SPB   CPYE;
      +     -1;
      T     #dwTmp;
      L     DBB [AR1,P#0.0];
      T     DIB [AR2,P#0.0];
      +AR1  P#1.0;
      +AR2  P#1.0;
      SPA   SCPY;
CPYE: NOP   0;

// dekodieren

ign:  NOP   0;
      SPA   ret;

NETWORK
TITLE =

ret:  BE    ;

NETWORK
TITLE =
//1. PC_RecvTeleFlag aktualisieren, weil Telegramm empfangen
//2. Wenn Partner wiederkommt (offline -> online), LastRecvDataPacketId auf -1
//setzen
rrrr: NOP   0;
      L     #wPcStationNumber;
      +     -1;
      L     1;
      SLD   ;
// Akku1 == 2 ^ (PCStationNumber - 1)
      LAR1  ; // Temp-Akku
      L     "abvspu_DB_UDP".PC_RecvTeleFlag;
      OD    ;
      T     "abvspu_DB_UDP".PC_RecvTeleFlag;
      TAR1  ; // Temp-Akku
// Akku1 == 2 ^ (PCStationNumber - 1)


      L     "abvspu_DB_UDP".PC_ONLINE;
      UD    ;
      SPP   a001;

// offline->online (LastRecvDataPacketId := -1)

      TAR1  #dwTmp;
      L     #wPcStationNumber;
      L     1;
      -D    ;
      L     32;
      *D    ;
      L     "abvspu_DB_UDP".dPtrLastRecvDataPacketId; // Zeiger auf PC-PacketId-Variablen im DB190
      +D    ;
      LAR1  ;

      AUF   "abvspu_DB_UDP";
      L     L#-1;
      T     DBD [AR1,P#0.0];

      LAR1  #dwTmp;

a001: TAR1  ; // Temp-Akku
      L     "abvspu_DB_UDP".PC_ONLINE;
      OD    ;
      T     "abvspu_DB_UDP".PC_ONLINE;

      L     #wReturnMark;
      SPL   unkn;
      SPA   r000;
      SPA   r001;
unkn: BE    ; // not possible

NETWORK
TITLE =

tolo: NOP   0; // packet id too low

      L     L#-1;
      T     "abvspu_DB_UDP".dwLastSentDataPacketId;
      TAD   ;
      T     "abvspu_DB_UDP".SendTeleHeader.PacketId;

      L     DW#16#FFFE;
      L     "abvspu_DB_UDP".wUDPPacketSize;
      /D    ;
      L     1;
      -D    ;
      T     "abvspu_DB_UDP".wPacketLastReadNdx;
      T     "abvspu_DB_UDP".wPacketLastWriteNdx;

      L     "abvspu_DB_UDP".wUDP_DB; // DbNo UDP-Sendepakete
      T     #wDBNo;
      AUF   DB [#wDBNo];

// clear DB191:
      L     -1;
      T     #wTmp;
lp:   NOP   0;
      L     #wTmp;
      +     1;
      T     #wTmp;
      L     DBLG;
      >=I   ;
      SPB   ftg;
      LAR1  P#DBX 0.0;
      TAK   ;
      SLD   3;
      +AR1  ;
      L     0;
      T     B [AR1,P#0.0];
      SPA   lp;

ftg:  NOP   0;
      L     0;
      T     "abvspu_DB_UDP".dwSendBusy;

      L     "spuDB_CFG".D_52; // (HilfsDB1) DB195.DBW104
      T     #wTmp;
      AUF   DB [#wTmp];
      SET   ;
      =     DBX  171.0; // Generalabfrage einleiten
      =     "abvspu_DB_GLO".Tele_DT.bSend;
      CALL "abvspu_RESET_AEND_DB" ;
      BE    ;

END_FUNCTION

FUNCTION "abvspu_INIT" : VOID
TITLE = Initialisierung Gesamtsystem
//
// Funktion:
// ---------
//
// History:
// --------
// 08-Nov-2004
// - check the compatibility no of spu-database
// 18-Apr-2001 (fixed)
// - Zykluszaehler "Senden" auf <max-1> setzen
// 18-Okt-2001 (added)
// - Levelcounter zuruecksetzen
//
AUTHOR : ab_rfe
FAMILY : AbvSpu
NAME : InitSpu
VERSION : 2.1


VAR_TEMP
  act_time : TIME ;
  wHelp1DB : WORD ;
  wDB : WORD ;
  iCnt : INT ;
END_VAR
BEGIN
NETWORK
TITLE =Restart-Flag
//restart flag
      SET   ;
      =     "abvspu_DB_GLO".bRestart;

//clear level-counter
      AUF   "abvspu_DB_GLO";
      LAR1  "abvspu_DB_GLO".AR_LvlCnt;
      L     16;
NEXT: T     #iCnt;
      L     0;
      T     DBW [AR1,P#0.0];
      +AR1  P#2.0;
      L     #iCnt;
      LOOP  NEXT;

      L     "spuDB_CFG".D_52; // DB195.DBW104
      T     #wHelp1DB;

//Anlaufkennung AbvSpu ruecksetzen;
      L     W#16#FFFF;
      T     "spuDB_CFG".D_80; // DB195.DBW160
//Anlaufkennung SAPI ruecksetzen;
      T     "spuDB_CFG".D_93; // DB195.DBW186

//Check compatibility number
      L     "abvspu_DB_VERSION".SPU_COMPATIBILITY_NUMBER; // spu compatibility number
      L     "spuDB_CFG".D_18; // spu-database compatibility number (AvET)
      ==D   ;
      SPB   a001;
      L     W#16#FF01; // Fehler: Spu-Database nicht kompatibel
      BEA   ;

a001: NOP   0;
      CALL "abvspu_DB_CHECK" ;
      L     W#16#0;
      ==I   ;
      SPB   OKAY;
      BEA   ;

OKAY: NOP   0;
//Anlaufkennung AbvSpu setzen;
      L     0;
      T     "spuDB_CFG".D_80; // DB195.DBW160

      L     "spuDB_CFG".D_90; // DB195.DBW180 (DB-Nr. SAPI)
      L     0;
      ==I   ;
      SPB   NSAP;
//Initialisierung SAPI/BSND/UDP-Schnittstelle
      CALL "abvspu_UDP_INIT" ;
NSAP: NOP   0;

      L     "spuDB_CFG".D_10; // DB195.DBW20 (1st ZDB)
      T     #wDB;
      CALL "abvspu_InitPvObj" (// Initialisierung PV-Obj
           DBXK                     := #wDB);

// Zeitstempel eintragen
      L     0;
      T     "abvspu_DB_GLO".Time_Tck_Prev;

      CALL "abvspu_100MS_TS" ;

      SET   ;
      AUF   DB [#wHelp1DB];
//hk: nicht bei UDP, Generalabfrage wird von kleinster OS ausgelöst.
      =     DBX  171.0; // Generalabfrage einleiten

// Eintragszaehler in AenderungsDBs ruecksetzen;
      CALL "abvspu_RESET_AEND_DB" ;// DB <INIT_VAL>

// Anfangswerte
      L     "spuDB_CFG".D_77; // DB195.DBW154
      L     0;
      ==I   ;
      SPB   NOIV;
      TAK   ;
      CALL "abvspu_INITVALUES" ;

// Zykluszaehler "Senden" auf <max-1> setzen;
NOIV: NOP   0;
      L     "spuDB_CFG".D_95; // DB195.DBW190
      DEC   1;
      T     "spuDB_CFG".D_96; // DB195.DBW192 - DB <XPadt-AutoClear>

      SPA   NOXP;

//xpadt-specials;
//
      L     "spuDB_CFG".D_78; // DB195.DBW156
      L     0;
      ==I   ;
//Initialisiere DB_GLOB (xpadt)
      SPB   NOXP;
      SET   ; //"DB_GLOB"._XpdTrue
      =     DB100.DBX    0.0; //"DB_GLOB"._XpdReset
      =     DB100.DBX    0.2;

//Vorbesetzungen
NOXP: NOP   0;
      L     0;
      T     "abvspu_DB_GLO".MaxTimeSend1Ms;
      CLR   ;

      =     "abvspu_DB_GLO".bTimeSend; // Uhrzeitabgleich
      L     "spuDB_CFG".D_83; // DB195.DBW166
      L     0;
      ==I   ;
//Initialisiere DB_GLO (TimeSync)
      SPB   NOTS;
      TAK   ;
      L     1000;
      *D    ;
      T     "abvspu_DB_GLO".MaxTimeSend1Ms;
      SET   ;
      =     "abvspu_DB_GLO".bTimeSend;
NOTS: NOP   0;
END_FUNCTION

FUNCTION "abvspu_CP_RECV" : VOID
TITLE = CP_RECV
//
//CP-Recv
//
// Historie
// # 08_Nov_2006 (added)
// - Receive multiple telegrams from FC191 in one OB1 cycle (up to 10)
AUTHOR : ab_rfe
FAMILY : AbvSpu
NAME : CP_RECV
VERSION : 2.0


VAR_TEMP
  wRecvDB : WORD ;
  bNewData : BOOL ;	//New Data Received in FC191 (TRUE = Yes)
  wRcveAttCnt : WORD ;	//Attempt Counter for 'Receive Data fromFC191'
END_VAR
BEGIN
NETWORK
TITLE = CP_Recv
//UDP-Recv;

//***********
//uHo
      L     0;
      T     #wRcveAttCnt; // Init counter for receive attempts
//***********



recv: CALL "abvspu_UDP_RECV" (
           RET_VAL                  := #bNewData);


//AbvSpu_Recv;
      CALL "abvspu_RECV_DB_1" ;


//***********
//uHo
      UN    #bNewData;
      BEB   ; // End receiving for this OB1 cycle, if there is nthing more to receive

      L     #wRcveAttCnt;
      L     1;
      +I    ; // Increment counter for receive attempts
      T     #wRcveAttCnt;

      L     40;
      <I    ;
      SPB   recv; // repeat with up to 40 attempts in total to receive a telegram
//***********
END_FUNCTION

FUNCTION "abvspu_Work_AMP" : VOID
TITLE =Bearbeitung Analog-MS
//
// History:
// --------
// 06-Nov-2004
// - Struktur DB180/181 erweitert (UndefGrp)
//
AUTHOR : ab_rfe
FAMILY : AbvSpu
NAME : Work_AMP
VERSION : 1.1


VAR_TEMP
  wDB : WORD ;	//DB-Nummer
  wObj : WORD ;	//Objektnummer
  wOpdType : WORD ;	//Operandentyp
  wHWM : WORD ;	//Hardwaremodul
  f32bitSignal : BOOL ;	//32bit-Eingangssignal
  dPtr_OpdAddr : DWORD ;	//Operandenadresse im Zeigerformat (zum Laden in AR)
  dARZ : DWORD ;	//Adressregister Zeigerliste
  dAnzMS : DWORD ;	//Anzahl MS in Zeigerliste
  iFC_obj : INT ;	//Parameter 1 (Objektnummer)
  iFC_type : INT ;	//Parameter 2 (Typkennung)
  dFC_signal : DWORD ;	//Parameter 3 (Signalwert)
  dFC_out_value : WORD ;
  bFC_out_flag : BOOL ;
  wFC_MSD_DbNo : WORD ;	//DB-Nummer MS-Datenfeld
  wFC_MSD_Offset : WORD ;	//Byteoffset MS-Datenfeld
  wUndefGrp : WORD ;	//Undefined Group
  wTmp1 : WORD ;
END_VAR
BEGIN
NETWORK
TITLE =AnaMS

      L     "spuDB_CFG".D_0; //DB195.DBW0 (DB-Nummer 'Zeigerliste Ana-MS')
      L     0;
      ==I   ;
      BEB   ;

      TAK   ;
      T     #wDB;
      L     "spuDB_CFG".D_15; //DB195.DBW30 (Objektnummer Ana-MS, 1st)
      T     #wObj;

      L     L#0;
      T     #dARZ;

      L     DW#16#FFFF; //Endlosschleife, Abbruch mit Endekennung
NEXT: T     #dAnzMS;

      CLR   ;
      =     #bFC_out_flag;

      L     #dARZ;
      LAR1  ;

      AUF   DB [#wDB]; //Zeigerliste öffnen

      L     DBW [AR1,P#0.0]; //MS-Datenfeld (DB-Nummer)
      L     W#16#FFFF; //Endekennung Zeigerliste
      ==D   ;
      SPB   ENDE;
      TAK   ;
      L     0;
      ==D   ; //spare record
      SPB   a002; //next record

      TAK   ;
      T     #wFC_MSD_DbNo;

      L     DBW [AR1,P#2.0]; //MS-Datenfeld (DW-Offset)
      T     #wFC_MSD_Offset;

      L     DBW [AR1,P#10.0]; //Undefined Group
      T     #wUndefGrp;

      L     DBB [AR1,P#5.0]; //S7-Info (DR=Hardwaremodul)
      T     #wHWM;
      L     17;
      ==I   ;
      =     #f32bitSignal;

      L     DBW [AR1,P#6.0]; //Opd.Bereich (DB-Byteoffset bzw. PEW-/MW-Adresse)
      SLD   3; //mal8
      T     #dPtr_OpdAddr;

      L     DBB [AR1,P#4.0]; //S7-Info (DL=Operandentyp)
      T     #wOpdType;

      SPL   SPL1;
      SPA   TY_0; //0=Eingang
      SPA   TY_1; //1=Merker
      SPA   TY_2; //2=DB
      SPA   TY_3; //3=Ausgang

SPL1: NOP   0; //>3 (unzulässig)
      SPA   a002;

TY_0: NOP   0; //Eingang (PEWx)
      L     #wHWM;
      T     #iFC_type;

      LAR2  #dPtr_OpdAddr;

      L     PEW [AR2,P#0.0];
      T     #dFC_signal;

      SPA   a001;

TY_1: NOP   0; //Merkerbereich
      L     #wHWM;
      T     #iFC_type;

      UN    #f32bitSignal;
      SPB   M_16;
      NOP   0;
      LAR2  #dPtr_OpdAddr;
      L     MD [AR2,P#0.0];
      SPA   M_XX;
M_16: NOP   0;
      LAR2  #dPtr_OpdAddr;
      L     MW [AR2,P#0.0];
M_XX: NOP   0;
      T     #dFC_signal;

TY_2: NOP   0; //DB-Adresse

      L     #wHWM;
      T     #iFC_type;

      L     DBW [AR1,P#8.0]; //DB-Operandenbereich (DB-Nummer)
      T     #wTmp1;
      AUF   DI [#wTmp1];
      LAR2  #dPtr_OpdAddr;

      UN    #f32bitSignal;
      SPB   D_16;
      NOP   0;
      L     DID [AR2,P#0.0];
      SPA   D_XX;
D_16: NOP   0;
      L     DIW [AR2,P#0.0];
D_XX: NOP   0;
      T     #dFC_signal;

      SPA   a001;

TY_3: NOP   0; //Ausgang (PAWx)

      L     256;
      T     #iFC_type;

a001: NOP   0;
      L     #wObj;
      T     #iFC_obj;

//      TAR2  #dAR2                       //AR2 retten

      CALL "abvspu_AMP" (
           OBJ                      := #iFC_obj,
           _TYPE                    := #iFC_type,
           IN_VALUE                 := #dFC_signal,
           MSD_DBNO                 := #wFC_MSD_DbNo,
           MSD_OFFSET               := #wFC_MSD_Offset,
           UNDEF_GRP                := #wUndefGrp,
           OUT_VALUE                := #dFC_out_value,
           OUT_FLAG                 := #bFC_out_flag);


//      LAR2  #dAR2                       //AR2 restaurieren

      UN    #bFC_out_flag;
      SPB   a002;

//Ausgangs-MS (PAWx)
      LAR2  #dPtr_OpdAddr;
      L     #dFC_out_value;
      T     PAW [AR2,P#0.0];

a002: NOP   0;

      LAR1  #dARZ;
      +AR1  P#12.0; //nächstes Datenfeld in Zeigerliste
      TAR1  #dARZ;

      L     #wObj; //nächste Objektnummer
      L     1;
      +D    ;
      T     #wObj;

      L     #dAnzMS;
      LOOP  NEXT;

ENDE: NOP   0;

END_FUNCTION

FUNCTION "abvspu_UDP_SEND" : VOID
TITLE = UDP_SEND
//
// Funktion:
// - Aenderungs-DBs in Sendekacheln schreiben
//
// Historie
// # 23-Jan-2006 (added)
// - Time master ( DB195.DBX  165.0 == 1 ) sendet Uhrzeit-Synchr.-Tele, wenn die
//   projektierte Anzahl von Zykluszeiten "abvspu_DB_GLO".wTimeSyncCycleCount)
//   abgelaufen ist
// # 29-Jun-2005 (fixed)
// - nach Setzen des Send-GA-Bit (DBX 171.0 des Hilfs-DB) zusätzlich
//   "abvspu_DB_GLO".Tele_DT.bSend setzen (Date/Time senden)
// # 22-Apr-2004 (added)
// - Fallunterscheidung CPU 300/400
// # 24-Mar-2004 (fixed)
// - NW <Freie Verbindungen ermitteln>
// - Parameter <LADDR> von W#16#3FFD nach "abvspu_DB_UDP".wLAddr[1]
// # 26-Jan-2004 (fixed)
// # 16-Okt-2003 (new)
//
//
AUTHOR : ab_rfe
FAMILY : AbvSpu
NAME : UDP_SEND
VERSION : 2.5


VAR_TEMP
  anyPtrSend : ANY ;	//ANY-Pointer, der auf Send-UDP-Packet zeigt
  wUDP_ControlDB : WORD ;	//DB 190 (Kommandobereich)
  wUDP_DataDB : WORD ;	//DB 191 (Datenpakete)
  wStsDmp : WORD ;
  wStsAmp : WORD ;
  wValDmp : WORD ;
  wValAmp : WORD ;
  wValPv : WORD ;
  wStrPv : WORD ;
  wDbNull : WORD ;
  wChgPara : WORD ;
  wChgLmt : WORD ;
  wDateTimeDB : WORD ;
  wOldTeleType : WORD ;	// Telegrammtyp
  wCurrentTimeStamp : WORD ;
  wAnzPC : WORD ;
  snd_len : INT ;
  snd_done : BOOL ;
  snd_error : BOOL ;
  snd_status : WORD ;
  iTmp : INT ;
  iAnzConnections : INT ;
  iActConnection : INT ;
  dwMaske : DWORD ;
  dwAct : DWORD ;
  bNextSrcDB : BOOL ;
  bNewSrcDB : BOOL ;
  bNewTeleHeader : BOOL ;
  bNewTimeStamp : BOOL ;
  bNextTile : BOOL ;
  bTileInUse : BOOL ;
  bWrite2Logfile : BOOL ;
  wTileUsedBytes : WORD ;
  wTileTeleHeadLen : WORD ;
  wTileSize : WORD ;
  yChgType : BYTE ;
  wDb : WORD ;
  wDbMaxPlus1 : WORD ;
  wDbNo : WORD ;
  wSrcDb : WORD ;
  wTeleType : WORD ;
  wTileTeleNettoLen : WORD ;
  wSrcRecLen : WORD ;
  wSrcRecOffs : WORD ;
  wSrcAnzDF : WORD ;
  wTimeStamp : WORD ;
  wRS : WORD ;
  wRT : WORD ;
  wOldTimeStamp : WORD ;
  dStr_Ptr : DWORD ;
  wStr_DB : WORD ;
  wStr_LenB : WORD ;
  wStr_LenW : WORD ;
  bOddStr : BOOL ;
  dTmpAR1 : DWORD ;
  strcpy_AnzB : WORD ;
  wCopyAnzWords : WORD ;
  wQ_Offs : WORD ;
  wZ_Offs : WORD ;
  wMaxPacketCount : WORD ;
  wActPacketCountWrite : WORD ;
  wPacketActWriteNdx : WORD ;
  wActPacketCountRead : WORD ;
  wPacketActReadNdx : WORD ;
  wPacketCountRollbackMax : WORD ;
  dPtrUDPHeader : DWORD ;
  dPtrUDPAct : DWORD ;
  dPtrUDPNettoDataHeader : DWORD ;
  dArSrcDb_0 : DWORD ;	// Adressregister AendDB (temporaer)
  dArSrcDb_x : DWORD ;	// Adressregister AendDB (temporaer)
  bSendNettoData : BOOL ;
  wTmp1 : WORD ;
  iTmpLength : INT ;
  dwTmpPacketId : DWORD ;
  wTmpUDPLogDBNo : WORD ;
  dwTmpAR2 : DWORD ;
END_VAR
BEGIN
NETWORK
TITLE = Initialisierung

      U     DB195.DBX  186.0; // UDP-Initialisierung okay?
      BEB   ;

      U     DB195.DBX  165.0; // time master ?
      SPBN  slav;

      L     "abvspu_DB_GLO".wActTimeSyncCycle;
      +     1;
      T     "abvspu_DB_GLO".wActTimeSyncCycle;
      L     "abvspu_DB_GLO".wTimeSyncCycleCount;
      <I    ;
      SPB   slav;
      L     0;
      T     "abvspu_DB_GLO".wActTimeSyncCycle;
      CALL "abvspu_UDP_SendRecvDT" (
           bSend                    := TRUE);// senden


slav: L     "abvspu_DB_UDP".wUDPLogDBNo;
      L     0;
      <>D   ;
      =     #bWrite2Logfile;

      CLR   ;
      =     #bSendNettoData;

      L     "abvspu_DB_UDP".wUDP_DB; // DB 191
      T     #wUDP_DataDB;

      L     "abvspu_DB_GLO".TimeStamp; // Zeitstempel aus DB_GLO
      T     #wCurrentTimeStamp;

// Anzahl PCs;
      L     "spuDB_CFG".D_81; // DB195.DBW162
      T     #wAnzPC;
// DB-Nr. AbvSpu-Aenderungsbausteine;
      L     "spuDB_CFG".D_44; // DB195.DBW88
      T     #wStsDmp; // Zustands-Aenderung DMP
      L     "spuDB_CFG".D_45; // DB195.DBW90
      T     #wStsAmp; // Zustands-Aenderung AMP
      L     "spuDB_CFG".D_46; // DB195.DBW92
      T     #wValDmp; // Messwert-Aenderung DMP
      L     "spuDB_CFG".D_47; // DB195.DBW94
      T     #wValAmp; // Messwert-Aenderung AMP
      L     "spuDB_CFG".D_49; // DB195.DBW98
      T     #wValPv; // Messwert-Aenderung PV
      L     "spuDB_CFG".D_50; // DB195.DBW100
      T     #wStrPv; // String-Aenderung PV
      L     0; // frei
      T     #wDbNull;
      L     "spuDB_CFG".D_60; // DB195.DBW120
      T     #wChgPara; // Quittierung Nachparametrieren
      L     "spuDB_CFG".D_48; // DB195.DBW96
      T     #wChgLmt; // Dynamisches Limit
      L     196;
      T     #wDateTimeDB; // Datum/Uhrzeit
      L     "spuDB_CFG".D_90; // DB195.DBW180
      T     #wUDP_ControlDB; // DB-Nr. UDP-ControlDB

      L     "abvspu_DB_UDP".wCountConnections;
      T     #iAnzConnections;
NETWORK
TITLE =Freie Verbindungen ermitteln
// ANY (anyPtrSend) ab LB 0 teilweise versorgen:
      L     W#16#1002;
      T     LW     0;

      L     "abvspu_DB_UDP".wUDPPacketSize; //1048
      T     LW     2;

      L     #wUDP_DataDB;
      T     LW     4;


      L     0;
      T     "abvspu_DB_UDP".dwSndInfo_ConnectionFree[1];

      L     1;
      T     #dwMaske;

      L     #iAnzConnections;
nxid: T     #iTmp;
      L     #iAnzConnections;
      TAK   ;
      -I    ;
      L     "abvspu_DB_UDP".wFirstConnection;
      +I    ;
      T     #iActConnection;

      L     "abvspu_DB_UDP".dwConnectionAvailable[1];
      L     #dwMaske;
      UD    ;
      SPZ   nxcn;

//      L     "abvspu_DB_UDP".wUDPPacketSize
//      T     #iTmpLength

//      SPA   nbsy

////////////////////////////

      L     #iActConnection;
      L     "abvspu_DB_UDP".wFirstConnection;
      -D    ;
      L     1;
      SLD   ;

      L     "abvspu_DB_UDP".dwSendBusy;
      UD    ;
      U     ==0;
      SPB   nbsy;

      LAR2  "abvspu_DB_UDP".dPtrLastSentDataLength;
      L     #iActConnection;
      L     "abvspu_DB_UDP".wFirstConnection;
      -D    ;
      SLD   4;
      +AR2  ;
      L     W [AR2,P#0.0];
//      T     LW     2                    // Längenangabe aus anyPtrSend
      T     #iTmpLength;


      LAR2  "abvspu_DB_UDP".dPtrLastDataPtr;
      L     #iActConnection;
      L     "abvspu_DB_UDP".wFirstConnection;
      -D    ;
      SLD   5;
      +AR2  ;
      L     D [AR2,P#0.0];
      T     LD     6; // Ber.übergr.Zeiger aus anyPtrSend

      L     LW     0;
      L     LW     2;
      L     LW     4;
      L     LD     6;

      CALL "abvspu_AGxSEND" (
           ACT                      := FALSE,
           ID                       := #iActConnection,
           LADDR                    := "abvspu_DB_UDP".wLAddr[1],
           SEND                     := #anyPtrSend,
           LEN                      := #iTmpLength,
           DONE                     := #snd_done,
           ERROR                    := #snd_error,
           STATUS                   := #snd_status);

      SPA   xbsy;


///////////////////////////





nbsy: NOP   0;
      L     "abvspu_DB_UDP".wUDPPacketSize;
      T     #iTmpLength;

      CALL "abvspu_AGxSEND" (
           ACT                      := FALSE,
           ID                       := #iActConnection,
           LADDR                    := "abvspu_DB_UDP".wLAddr[1],
           SEND                     := "abvspu_DB_UDP".LifeSignTele,
           LEN                      := #iTmpLength,
           DONE                     := #snd_done,
           ERROR                    := #snd_error,
           STATUS                   := #snd_status);

xbsy: NOP   0;
//      L     #snd_status
//      L     W#16#8183
//      <>D
//      SPB   avai
      SPA   avai;

      L     "abvspu_DB_UDP".dwConnectionAvailable[1];
      L     #dwMaske;
      INVD  ;
      UD    ;
      T     "abvspu_DB_UDP".dwConnectionAvailable[1];
      SPA   nxcn;

avai: L     #snd_status;
      L     W#16#7000;
      ==D   ;
      SPB   free;

      UN    #snd_error;
      SPB   noer;

      L     "abvspu_DB_UDP".dwSndInfo_Error[1];
      L     #dwMaske;
      OD    ;
      T     "abvspu_DB_UDP".dwSndInfo_Error[1];
      SPA   nxcn;

noer: L     #snd_status;
      L     W#16#8181;
      ==D   ;
      SPB   nxcn;

free: NOP   0;
      L     "abvspu_DB_UDP".dwSndInfo_ConnectionFree[1];
      L     #dwMaske;
      OD    ;
      T     "abvspu_DB_UDP".dwSndInfo_ConnectionFree[1];

      L     #dwMaske;
      INVD  ;
      L     "abvspu_DB_UDP".dwSendBusy;
      UD    ;
      T     "abvspu_DB_UDP".dwSendBusy;

nxcn: L     #dwMaske;
      SLD   1;
      T     #dwMaske;

      L     #iTmp;
      LOOP  nxid;


      L     DW#16#FFFE;
      L     "abvspu_DB_UDP".wUDPPacketSize;
      /D    ;
      T     #wMaxPacketCount; // == 62

      L     DB195.DBB  105; // HilfsDB_1
      T     #iTmp;
      AUF   DB [#iTmp];
      U     DBX  171.0; // Generalabfrage läuft
      SPB   v001;

      L     1;
      L     "spuDB_CFG".D_96; //Zykluszaehler (DB195.DBW192)
      +I    ;
      L     "spuDB_CFG".D_96; //Zykluszaehler (DB195.DBW192)
      L     "spuDB_CFG".D_95; //Sendezyklus (DB195.DBW190)
      MOD   ;
      L     0;
      <>I   ;
      SPB   DOXX;

v001: NOP   0;
NETWORK
TITLE =Änderungsdatenbausteine entsorgen

      U     "abvspu_DB_UDP".bRecvRollbackRequest;
      SPB   roll;
      U     "abvspu_DB_UDP".bDoRollback; // für Testzwecke
      SPB   roll; // rollback geht vor Entsorgen der Änderungs-DBs

// ######################################################################

// (R-S-W) + (W >= R ? 62 : 0)
      L     "abvspu_DB_UDP".wPacketLastReadNdx;
      L     "abvspu_DB_UDP".wPacketLastWriteNdx;
      -D    ;
      L     "abvspu_DB_UDP".wSentPackets4Rollback;
      -D    ;
      T     #wActPacketCountWrite;
      L     "abvspu_DB_UDP".wPacketLastWriteNdx;
      L     "abvspu_DB_UDP".wPacketLastReadNdx;
      <D    ;
      SPB   tmp1;
      L     #wActPacketCountWrite;
      L     62;
      +D    ;
      T     #wActPacketCountWrite;
tmp1: L     #wActPacketCountWrite;
      L     0;
      ==D   ;
      SPB   QSND; // send UDP-Data ?

      L     "abvspu_DB_UDP".wPacketLastWriteNdx;
      L     1;
      +D    ;
      L     #wMaxPacketCount;
      MOD   ;
      T     #wPacketActWriteNdx; // aktueller Schreibindex

      L     "abvspu_DB_UDP".wUDPPacketSize; //1048
      L     24; // UDP-Header size
      -D    ;
      T     #wTileSize;
      L     8;
      T     #wTileTeleHeadLen;
// Status- und Messwertaenderungen;
// Schleifenzaehler (10 DBs);
      L     1;
      T     #wDb;
      L     11; //10+1;
      T     #wDbMaxPlus1;
// Aktuelle DB-Nr. laden;
      L     "abvspu_DB_UDP".wActSrcDBNo;
      T     #wDbNo;
// Aktuelle Kachel-Nr. laden;
//    L     "abvspu_DB_UDP".FREE2[2];

      CLR   ;
      =     #bTileInUse;

LOP1: NOP   0; //alle AenderungsDBs bearbeiten

      CLR   ;
      =     #bNextSrcDB;
      =     #bNewSrcDB;

      L     0;
      T     #yChgType;

      L     DW#16#FFFFFFFF;
      T     #dArSrcDb_x;
      T     #dArSrcDb_0;

      L     #wDb;
      L     #wDbMaxPlus1;
      ==I   ;
      SPB   X000; //alle DBs entsorgt;

      L     #wDbNo;
// Sprungverteiler <AenderungsDBs>
      SPL   SPL1;
      SPA   X000;
      SPA   STS1; // Zustand BMS
      SPA   STS2; // Zustand AMS
      SPA   PVAL; // PV-Messwert
      SPA   PSTR; // PV-String
      SPA   VAL1; // Messwert BMS
      SPA   VAL2; // Messwert AMS
      SPA   ADBX; // frei
      SPA   PAR1;
      SPA   DYLI;
      SPA   DATI;
SPL1: SPA   X000;
X000: NOP   0;
//alle DBs entsorgt;
      SPA   ENDE;
STS1: NOP   0;
//1. Aenderungs-DB (Zustand BMS);
      L     1;
      T     #yChgType;
      L     #wStsDmp;
      T     #wSrcDb;
// Telegrammtyp Zustandsaenderung (MS-bin/ana);
      L     4;
      T     #wTeleType;
// Telegrammlaenge (bytes) in UDP-Packet
      L     8;
      T     #wTileTeleNettoLen;
// Datensatzlaenge (w);
      L     5;
      T     #wSrcRecLen;
      SLW   4;
      T     #wSrcRecOffs;
      SPA   WORK;
STS2: NOP   0;
//2. Aenderungs-DB (Zustand AMS);
      L     1;
      T     #yChgType;
      L     #wStsAmp;
      T     #wSrcDb;
// Telegrammtyp Zustandsaenderung XMP/XPO;
      L     4;
      T     #wTeleType;
// Telegrammlaenge (bytes) in Kachel
      L     8;
      T     #wTileTeleNettoLen;
// Datensatzlaenge;
      L     5;
      T     #wSrcRecLen;
      SLW   4;
//        NEGI;
      T     #wSrcRecOffs;
      SPA   WORK;
PVAL: NOP   0;
//3. Aenderungs-DB (PV-Messwert);
      L     6;
      T     #yChgType;
      L     #wValPv;
      T     #wSrcDb;
// Telegrammtyp PV-Messwert;
      L     5;
      T     #wTeleType;
// Telegrammlaenge (bytes) in Kachel
      L     6;
      T     #wTileTeleNettoLen;
// Datensatzlaenge;
      L     5;
      T     #wSrcRecLen;
      SLW   4;
//        NEGI;
      T     #wSrcRecOffs;
      SPA   WORK;
PSTR: NOP   0;
//4. Aenderungs-DB (PV-String);
      L     7;
      T     #yChgType;
      L     #wStrPv;
      T     #wSrcDb;
// Telegrammtyp Zustandsaenderung XMP/XPO;
      L     18;
      T     #wTeleType;
// Telegrammlaenge (bytes) in Kachel
      L     8;
      T     #wTileTeleNettoLen;
// Datensatzlaenge;
      L     5;
      T     #wSrcRecLen;
      SLW   4;
//        NEGI;
      T     #wSrcRecOffs;
      SPA   WORK;
VAL1: NOP   0;
//5. Aenderungs-DB (Messwert BMS);
      L     2;
      T     #yChgType;
      L     #wValDmp;
      T     #wSrcDb;
// Telegrammtyp Messwertaenderung XMP/APO;
      L     5;
      T     #wTeleType;
// Telegrammlaenge (bytes) in Kachel
      L     6;
      T     #wTileTeleNettoLen;
// Datensatzlaenge;
      L     4;
      T     #wSrcRecLen;
      SLW   4;
//        NEGI;
      T     #wSrcRecOffs;
      SPA   WORK;
VAL2: NOP   0;
//6. Aenderungs-DB (Messwert AMS);
      L     2;
      T     #yChgType;
      L     #wValAmp;
      T     #wSrcDb;
// Telegrammtyp Messwertaenderung XMP/APO;
      L     5;
      T     #wTeleType;
// Telegrammlaenge (bytes) in Kachel
      L     6;
      T     #wTileTeleNettoLen;
// Datensatzlaenge;
      L     4;
      T     #wSrcRecLen;
      SLW   4;
//        NEGI;
      T     #wSrcRecOffs;
      SPA   WORK;
ADBX: NOP   0;
//7. Aenderungs-DB (frei);
      L     #wDbNull;
      T     #wSrcDb;
      SPA   WORK;
PAR1: NOP   0;
//8. Aenderungs-DB (Nachparametrierung);
      L     3;
      T     #yChgType;
      L     #wChgPara;
      T     #wSrcDb;
// Telegrammtyp Quittierung Nachparametrierung;
      L     16;
      T     #wTeleType;
// Telegrammlaenge (bytes) in Kachel
      L     12;
      T     #wTileTeleNettoLen;
// Datensatzlaenge;
      L     7;
      T     #wSrcRecLen;
      SLW   4;
//        NEGI;
      T     #wSrcRecOffs;
      SPA   WORK;
DYLI: NOP   0;
//9. Aenderungs-DB (Dynamischer Grenzwert);
      L     5;
      T     #yChgType;
      L     #wChgLmt;
      T     #wSrcDb;
// Telegrammtyp Dynamischer Grenzwert;
      L     12;
      T     #wTeleType;
// Telegrammlaenge (bytes) in Kachel
      L     10;
      T     #wTileTeleNettoLen;
// Datensatzlaenge;
      L     5;
      T     #wSrcRecLen;
      SLW   4;
//        NEGI;
      T     #wSrcRecOffs;
      SPA   WORK;
DATI: NOP   0;
//Datum/Uhrzeit;
      UN    "abvspu_DB_GLO".Tele_DT.bSend;
//        SPB ENDE;                // nothing to do
      SPB   NXDB;

      L     4;
      T     #yChgType;
      L     #wDateTimeDB;
      T     #wSrcDb;
//      SET
//      =     #bNewSrcDB
      UN    #bTileInUse;
      SPB   LOP2;
//aktuelle Kachel abschliessen
      LAR2  #dPtrUDPNettoDataHeader;
//Telegrammheader aktualisieren;
      L     #wRT;
      T     DIW [AR2,P#0.0]; // Anzahl Eintraege Sendekachel;
      L     #wOldTeleType;
      T     DIW [AR2,P#2.0]; // Telegrammtyp;
      L     #wOldTimeStamp;
      T     DID [AR2,P#4.0]; // Timestamp;
      SPA   SNDX;

WORK: NOP   0;
//AenderungsDB pruefen;
      L     #wSrcDb;
      L     0;
      ==I   ;
      SPB   NXDB; // DB nicht vorhanden
      AUF   DB [#wSrcDb]; // Aenderungs-DB oeffnen
      L     DBW    0; // Anzahl Datenfelder
      T     #wSrcAnzDF;
      L     0;
      ==I   ;
      SPB   NXDB; // keine Aenderungen eingetragen
      SET   ;
      =     #bNewSrcDB; // neuer AenderungsDB
      U     #bTileInUse;
      SPB   ASDB; // aktuelle Kachel verwenden
LOP2: NOP   0;
// freie Sendekachel beginnen;

      L     #wPacketActWriteNdx; // aktueller Schreibindex
      L     "abvspu_DB_UDP".wUDPPacketSize;
      *I    ;
      SLD   3;
      LAR2  ;
      TAR2  #dPtrUDPHeader;

      AUF   DI [#wUDP_DataDB];

      L     "abvspu_DB_UDP".SendTeleHeader.SenderId;
      T     DID [AR2,P#0.0];
      L     "abvspu_DB_UDP".SendTeleHeader.PacketId;

      TAD   ;
      L     L#1;
      +D    ;
      TAD   ;

      T     DID [AR2,P#4.0];
      T     "abvspu_DB_UDP".SendTeleHeader.PacketId;

      L     "abvspu_DB_UDP".SendTeleHeader.ReceiverId;
      T     DID [AR2,P#8.0];

      L     "abvspu_DB_UDP".SendTeleHeader.PacketType;
      T     DID [AR2,P#12.0];

      L     0; // UDP-Header (24 Bytes) exclusive!
      T     DID [AR2,P#16.0]; // total Packet length

      L     "abvspu_DB_UDP".SendTeleHeader.PartialPacketId;
      T     DID [AR2,P#20.0];

      +AR2  P#24.0;
      TAR2  #dPtrUDPNettoDataHeader;
      TAR2  #dPtrUDPAct;


// Aenderungs-DB entsorgen;

// Zeiger auf 1. Eintrag Nettodaten (ObjNo,...);
//      +AR2  P#8.0
      L     0;
//      L     #wTileTeleHeadLen           // 8 Bytes
      T     #wTileUsedBytes; // Anzahl Bytes in abData[1..1024]
//      L     #wTileTeleHeadLen           // 8 Bytes
//      SLD   3
//      +AR2
//      TAR2  #dPtrUDPNettoData

//Kachel-Eintragszaehler ruecksetzen;
      L     0;
      T     #wRT;

// Kachel in Bearbeitung;
      SET   ;
      =     #bTileInUse;

//wird gesetzt, wenn ein AenderungsDB entsorgt wurde
      U     #bNextSrcDB;
      SPB   LOP1; // naechster AenderungsDB
ASDB: NOP   0;

      AUF   DB [#wSrcDb];
      AUF   DI [#wUDP_DataDB];

//;
//Zustands-Aenderung (MS)
//------------------------;
//DW  0:Anzahl Datenfelder;
//DBW+0:ObjNo;
//DBW+2:Status;
//DBD+4:Messwert;
//DBW+8:Zeitstempel;
//;
//Messwert-Aenderung (MS)
//------------------------;
//DW  0:Anzahl Datenfelder;
//DBW+0:ObjNo;
//DBD+2:Messwert;
//DBW+6:Zeitstempel;
//;
//Messwert-Aenderung (PV)
//------------------------;
//DW  0:Anzahl Datenfelder;
//DBW+0:Station;
//DBW+2:ObjNo;
//DBD+4:Messwert;
//DBW+8:Zeitstempel;
//;
//String-Aenderung (PV)
//------------------------;
//DW  0:Anzahl Datenfelder;
//DBW+0:Station;
//DBW+2:ObjNo;
//DBW+4:Str_DB;
//DBD+6:Str_Ptr;
//;

//;
//Zustands-Aenderung;
//------------------;
//DW  0:Anzahl Datenfelder;
//DW  1:Telegrammtyp;
//DD  2:Zeitstempel (TOD);
//DWn+0:ObjNo;
//DWn+1:Status;
//;
//Messwert-Aenderung;
//------------------;
//DW  0:Anzahl Datenfelder;
//DW  1:Telegrammtyp;
//DD  2:Zeitstempel (TOD);
//DWn+0:ObjNo;
//DWn+1:Value;
//DWn+2:Value;
//;
//Sonderbehandlung bei Datum/Uhrzeit;
      L     #yChgType;
      L     4;
      ==I   ;
      SPB   L204;
      U     #bNewSrcDB;
      SPB   NSDB; // neuer AenderungsDB...
//AenderungsDB ist bereits in Bearbeitung (Kachelwechsel);
      LAR1  #dArSrcDb_x; // Zeiger AenderungsDB laden
      L     #yChgType;
      SPL   SPL2;
      SPA   L200;
      SPA   L201; //MS-Zustand
      SPA   L202; //MS-Messwert
      SPA   L203; //MS-Nachparametrieren
      SPA   L204; //Datum/Uhrzeit
      SPA   L205; //Dyn. Grenzwert
      SPA   L206; //PV-Messwert
      SPA   L207; //PV-String
SPL2: SPA   L200;
L200: NOP   0;
L201: NOP   0;
//Status-Aenderung;
      L     DBW [AR1,P#8.0]; // aktuellen Zeitstempel
      T     #wTimeStamp;
      SPA   LCPY;
L202: NOP   0;
//Messwert-Aenderung;
      L     DBW [AR1,P#6.0]; // aktuellen Zeitstempel
      T     #wTimeStamp;
      SPA   LCPY;
L203: NOP   0;
//Nachparametrieren;
      L     DBW [AR1,P#12.0]; // aktuellen Zeitstempel
      T     #wTimeStamp;
      SPA   LCPY;
L205: NOP   0;
//Dyn. Grenzwert;
      L     DBW [AR1,P#8.0]; // aktuellen Zeitstempel
      T     #wTimeStamp;
      SPA   LCPY;
L206: NOP   0;
//PV-Messwert;
      L     DBW [AR1,P#8.0]; // aktuellen Zeitstempel
      T     #wTimeStamp;
      SPA   LCPY;
L207: NOP   0;
//PV-String;
      L     #wCurrentTimeStamp; // aktuellen Zeitstempel
      T     #wTimeStamp;
      SPA   LCPY;
L204: NOP   0;
//Datum/Uhrzeit;
      LAR2  #dPtrUDPNettoDataHeader;

      +AR2  P#8.0;
      L     "abvspu_DB_GLO".Tele_DT.wYeMo;
      T     DIW [AR2,P#0.0];
      L     "abvspu_DB_GLO".Tele_DT.wDaHo;
      T     DIW [AR2,P#2.0];
      L     "abvspu_DB_GLO".Tele_DT.wMiSe;
      T     DIW [AR2,P#4.0];

// LTC-Korrekturwert
      L     "abvspu_DB_GLO".aLTC_Correction[1];
      T     DIB [AR2,P#6.0];
      L     "abvspu_DB_GLO".aLTC_Correction[2];
      T     DIB [AR2,P#7.0];
      L     "abvspu_DB_GLO".aLTC_Correction[3];
      T     DIB [AR2,P#8.0];
      L     "abvspu_DB_GLO".aLTC_Correction[4];
      T     DIB [AR2,P#9.0];
      L     "abvspu_DB_GLO".aLTC_Correction[5];
      T     DIB [AR2,P#10.0];
      L     "abvspu_DB_GLO".aLTC_Correction[6];
      T     DIB [AR2,P#11.0];

      L     0;
      T     DIW [AR2,P#12.0]; // Ende-Kennung

// Sendekachel fertig machen;

      L     #wTileTeleHeadLen;
      L     12; // Nettodatenlänge
      +D    ;
      T     #wTileUsedBytes;

      LAR2  #dPtrUDPHeader;
      L     #wTileUsedBytes;
      TAD   ;
      T     DID [AR2,P#16.0];

      LAR2  #dPtrUDPNettoDataHeader;
// Anzahl Eintraege Sendekachel;
      L     1;
      T     DIW [AR2,P#0.0];
// Telegrammtyp;
      L     "abvspu_DB_GLO".Tele_DT.wTeleType;
      T     DIW [AR2,P#2.0];
// Timestamp;
      L     L#0;
      T     DID [AR2,P#4.0];
      CLR   ;
      =     "abvspu_DB_GLO".Tele_DT.bSend;
      SET   ;
      =     #bTileInUse;
      SPA   NXDB;
NSDB: NOP   0;
//neuer AenderungsDB;
      CLR   ;
      =     #bNewSrcDB;
// Zeiger Aenderungs-DB;
      L     0;
      T     #dArSrcDb_0; // Zeiger auf Anzahl Eintraege
      L     1;
      SLD   4;
      LAR1  ; // Zeiger auf 1. Eintrag (DW 1)
      TAR1  #dArSrcDb_x;
      L     1;
      T     #wRS;
//;
//1. Zeitstempel aus neuem AenderungsDB laden;
//;
      L     #yChgType;
      SPL   SPL3;
      SPA   L300;
      SPA   L301; //MS-Zustand
      SPA   L302; //MS-Messwert
      SPA   L303; //MS-Nachparametrieren
      SPA   L300; //frei
      SPA   L305; //Dyn. Grenzwert
      SPA   L306; //PV-Messwert
      SPA   L307; //PV-String
SPL3: SPA   L300;
L300: NOP   0;
L301: NOP   0;
//Status-Aenderung;
      L     DBW [AR1,P#8.0]; // 1. Zeitstempel
      T     #wTimeStamp;
      SPA   a001;
L302: NOP   0;
//Messwert-Aenderung;
      L     DBW [AR1,P#6.0]; // 1. Zeitstempel
      T     #wTimeStamp;
      SPA   a001;
L303: NOP   0;
//Nachparametrieren;
      L     DBW [AR1,P#12.0]; // 1. Zeitstempel
      T     #wTimeStamp;
      SPA   a001;
L305: NOP   0;
//Dyn. Grenzwert;
      L     DBW [AR1,P#8.0]; // 1. Zeitstempel
      T     #wTimeStamp;
      SPA   a001;
L306: NOP   0;
//PV-Messwert;
      L     DBW [AR1,P#8.0]; // 1. Zeitstempel
      T     #wTimeStamp;
      SPA   a001;
L307: NOP   0;
//PV-String;
      L     #wCurrentTimeStamp;
      T     #wTimeStamp;
      SPA   a001;
a001: NOP   0;
      UN    #bTileInUse;
      SPB   LCPY;
//;
      CLR   ;
      =     #bNewTeleHeader;

      L     #wTeleType;
      L     #wOldTeleType;
      <>I   ;
      S     #bNewTeleHeader;

      L     #wTimeStamp;
      L     #wOldTimeStamp;
      <>I   ;
      S     #bNewTeleHeader;

      SPA   CHK1;
LCPY: NOP   0;
//;
//von AenderungsDB in Kachel kopieren;
//;
      CLR   ;
      =     #bNewTeleHeader;
// rfe, 26.01.04
      L     #wTileUsedBytes;
      L     0;
      ==D   ;
      S     #bNewTeleHeader;

CHK1: NOP   0;
//Zeitstempelvergleich
      CLR   ;
      =     #bNewTimeStamp;
      L     #yChgType;
      SPL   SPL4;
      SPA   L400;
      SPA   L401; // MS-Zustand
      SPA   L402; //MS-Messwert
      SPA   L403; //Nachparametrieren
      SPA   L400; //frei
      SPA   L405; //Dyn. Grenzwert
      SPA   L406; //PV-Messwert
      SPA   L407; //PV-String
SPL4: SPA   L400;
L400: NOP   0;
L401: NOP   0;
//Status-Aenderung;
      L     DBW [AR1,P#8.0];
      L     #wTimeStamp;
      <>I   ;
      S     #bNewTimeStamp;
      SPA   b000;
L402: NOP   0;
//Messwert-Aenderung;
      L     DBW [AR1,P#6.0];
      L     #wTimeStamp;
      <>I   ;
      S     #bNewTimeStamp;
      SPA   b000;
L403: NOP   0;
//Nachparametrieren;
      L     DBW [AR1,P#12.0];
      L     #wTimeStamp;
      <>I   ;
      S     #bNewTimeStamp;
      SPA   b000;
L405: NOP   0;
//Dyn. Grenzwert;
      L     DBW [AR1,P#8.0];
      L     #wTimeStamp;
      <>I   ;
      S     #bNewTimeStamp;
      SPA   b000;
L406: NOP   0;
//PV-Messwert;
      L     DBW [AR1,P#8.0];
      L     #wTimeStamp;
      <>I   ;
      S     #bNewTimeStamp;
      SPA   b000;
L407: NOP   0;
//PV-String;
      CLR   ;
      =     #bNewTimeStamp;
      SET   ;
      =     #bNewTeleHeader;
      SPA   b000;
b000: NOP   0;
      UN    #bNewTimeStamp;
      SPB   NTHD;
//neuer Zeitstempel;
      TAK   ;
      T     #wTimeStamp;
      SET   ;
      =     #bNewTeleHeader;
NTHD: NOP   0;
      UN    #bNewTeleHeader;
      SPB   TIFR;
//;
//Neuer Telegrammheader: Wechsel von Zeitstempel oder Telegrammtyp
//;
//aktuellen Telegrammheader aktualisieren;
//neuen Telegrammheader einrichten;
//;
//noch Platz in Kachel?
      L     #yChgType;
      L     7;
      <>I   ;
      SPB   k001; // kein PV-String
// Sonderbehandlung <PV-Strings>
      L     DBD [AR1,P#6.0]; // akku2=Str_Ptr
      T     #dStr_Ptr;
      L     DBW [AR1,P#4.0]; // akku1=Str_DB
      T     #wStr_DB;
      CALL "abvspu_GetPvStrLen" ;// akku1=Stringlänge in Bytes
      L     4;
      +D    ;
      T     #wTileTeleNettoLen;

k001: L     #wTileUsedBytes;
      L     #wTileTeleHeadLen; //neuer Telegrammheader
      +I    ;
      L     #wTileTeleNettoLen;
      +I    ;
      L     #wTileSize;
      >I    ;
      =     #bNextTile; // -> neue Kachel
      SPB   TCOP;
//;
//aktuelle Kachel weiterverwenden, neuer Telegrammheader;
//;
//aktuellen Telegrammheader versorgen;
      TAR2  #dPtrUDPAct; // Kachelzeiger retten;
      LAR2  #dPtrUDPNettoDataHeader;
      L     #wRT;
      T     DIW [AR2,P#0.0]; // Anzahl Eintraege Sendekachel;
      L     #wOldTeleType;
      T     DIW [AR2,P#2.0]; // Telegrammtyp;
      L     #wOldTimeStamp;
      T     DID [AR2,P#4.0]; // Timestamp;
//Kachel-Eintragszaehler ruecksetzen;
      L     0;
      T     #wRT;
//Kachelzeiger auf 1. Netto-Telegramm stellen;
      LAR2  #dPtrUDPAct;
      TAR2  #dPtrUDPNettoDataHeader; // Zeiger neuer Telegrammheader
      +AR2  P#8.0; // Zeiger 1. Netto-Telegramm
//Kachel-Bytezaehler um neuen Telegrammheader erhoehen;
      L     #wTileUsedBytes;
      L     #wTileTeleHeadLen;
      +I    ;
      T     #wTileUsedBytes;

      L     #yChgType;
      L     7;
      <>I   ;
      SPB   TCOP;

// Sonderbehandlung <PV-Strings>
      L     DBD [AR1,P#6.0]; // akku2=Str_Ptr
      T     #dStr_Ptr;
      L     DBW [AR1,P#4.0]; // akku1=Str_DB
      T     #wStr_DB;
      CALL "abvspu_GetPvStrLen" ;// akku1=Stringlänge in Bytes
      T     #wStr_LenB;
      TAK   ;
      T     #wStr_LenW;
      L     2;
      *I    ;
      +     4;
      T     #wTileTeleNettoLen; // Länge incl. StrLen+objno+Str_Nettodaten

      SPA   TCOP;
TIFR: NOP   0;
//noch Platz in Kachel?
      L     #yChgType;
      L     7;
      <>I   ;
      SPB   TYPX;
// Sonderbehandlung <PV-Strings>
      L     DBD [AR1,P#6.0]; // akku2=Str_Ptr
      T     #dStr_Ptr;
      L     DBW [AR1,P#4.0]; // akku1=Str_DB
      T     #wStr_DB;
      CALL "abvspu_GetPvStrLen" ;// akku1=Stringlänge in Bytes
      T     #wStr_LenB;
      TAK   ;
      T     #wStr_LenW;
      L     2;
      *I    ;
      +     4;
      T     #wTileTeleNettoLen; // Länge incl. StrLen+objno+Str_Nettodaten

TYPX: NOP   0; // Standard-Telegrammtypen
      L     #wTileUsedBytes;
      L     #wTileTeleNettoLen;
      +I    ;
      L     #wTileSize;
      >I    ;
      =     #bNextTile; // -> neue Kachel
TCOP: NOP   0;
      U     #bNextTile;
      SPB   EECP; // -> Kachel fertig machen und senden
//Netto-Telegramm in Kachel eintragen;
      SET   ;
      =     #bTileInUse;
      L     DBW [AR1,P#0.0]; // Objekt-Nr.
      T     DIW [AR2,P#0.0];

      L     #yChgType;
      SPL   SPL5;
      SPA   L500;
      SPA   L501; //MS-Zustand
      SPA   L502; //MS-Messwert
      SPA   L503; //Nachparametrieren
      SPA   L500; //frei
      SPA   L505; //Dyn. Grenzwert
      SPA   L506; //PV-Messwert
      SPA   L507; //PV-String
SPL5: SPA   L500;
L500: NOP   0;
L501: NOP   0;
//Status-Aenderung;
      L     DBW [AR1,P#2.0]; // Status
      T     DIW [AR2,P#2.0];
      L     DBD [AR1,P#4.0]; // Messwert
      T     DID [AR2,P#4.0];
      L     0;
      T     DID [AR2,P#8.0]; // Ende-Kennung
//Zeiger in Kachel und AenderungsDB weiterschalten;
      L     #wSrcRecOffs;
      +AR1  ; // naechster Eintrag Aenderungs-DB
      +AR2  P#8.0; // naechster Eintrag Sendekachel
      SPA   NCPY;
L502: NOP   0;
//Messwert-Aenderung;
      L     DBD [AR1,P#2.0]; // Messwert
      T     DID [AR2,P#2.0];
      L     0;
      T     DID [AR2,P#6.0]; // Ende-Kennung
//Zeiger in Kachel und AenderungsDB weiterschalten;
      L     #wSrcRecOffs;
      +AR1  ; // naechster Eintrag Aenderungs-DB
      +AR2  P#6.0; // naechster Eintrag Sendekachel
      SPA   NCPY;
L506: NOP   0;
//PV-Messwert;
      L     DBW [AR1,P#2.0]; // Objekt-Nr.
      T     DIW [AR2,P#0.0];
      L     DBD [AR1,P#4.0]; // PV-Messwert
      T     DID [AR2,P#2.0];
      L     0;
      T     DID [AR2,P#6.0]; // Ende-Kennung
//Zeiger in Kachel und AenderungsDB weiterschalten;
      L     #wSrcRecOffs;
      +AR1  ; // naechster Eintrag Aenderungs-DB
      +AR2  P#6.0; // naechster Eintrag Sendekachel
      SPA   NCPY;
L507: NOP   0;
//PV-String;

      L     #wStr_LenB;
      L     2;
      MOD   ;
      L     0;
      <>I   ;
      =     #bOddStr; // String ungerade

      L     #wTileTeleNettoLen;
      UN    #bOddStr;
      SPB   X900;
      +     -1;
X900: T     DIW [AR2,P#0.0]; // Länge
      L     DBW [AR1,P#2.0];
      T     DIW [AR2,P#2.0]; // Objekt-Nr.

      TAR1  #dTmpAR1; // Ptr -> Src_DB

      AUF   DB [#wStr_DB];
      LAR1  #dStr_Ptr;
      +AR1  P#2.0; // Ptr -> Nettodaten

      +AR2  P#4.0; //+2w
// *** strcpy *************************************************

      L     #wStr_LenB;
      T     #strcpy_AnzB; // Anzahl Bytes
SCPY: L     0;
      L     #strcpy_AnzB;
      ==I   ;
      SPB   CPYE;
      +     -1;
      T     #strcpy_AnzB;
      L     DBB [AR1,P#0.0];
      T     DIB [AR2,P#0.0];
      +AR1  P#1.0;
      +AR2  P#1.0;
      SPA   SCPY;
CPYE: NOP   0;

      UN    #bOddStr;
      SPB   EVEN;
      L     0;
      T     DIB [AR2,P#0.0];
      +AR2  P#1.0;

EVEN: NOP   0;
      AUF   DB [#wSrcDb];
      LAR1  #dTmpAR1; // Ptr -> Src_DB

      L     0;
      T     DID [AR2,P#0.0]; // Ende-Kennung

//Zeiger in Kachel und AenderungsDB weiterschalten;
      L     #wSrcRecOffs;
      +AR1  ; // naechster Eintrag Aenderungs-DB

      SPA   NCPY;

L503: NOP   0;
//Nachparametrieren;
      L     DBW [AR1,P#2.0]; // RelNo,Kennung
      T     DIW [AR2,P#2.0];
      L     DBW [AR1,P#4.0]; // Zeitverz. (kommend)
      T     DIW [AR2,P#4.0];
      L     DBW [AR1,P#6.0]; // Zeitverz. (gehend)
      T     DIW [AR2,P#6.0];
      L     DBD [AR1,P#8.0]; // Grenzwert
      T     DID [AR2,P#8.0];
      L     0;
      T     DID [AR2,P#12.0]; // Ende-Kennung
//Zeiger in Kachel und AenderungsDB weiterschalten;
      L     #wSrcRecOffs;
      +AR1  ; // naechster Eintrag Aenderungs-DB
      +AR2  P#12.0; // naechster Eintrag Sendekachel
      SPA   NCPY;
L505: NOP   0;
//Dyn. Grenzwert;
      L     DBW [AR1,P#2.0]; // RelNo,Kennung
      T     DIW [AR2,P#2.0];
      L     DBD [AR1,P#4.0]; // Grenzwert
      T     DID [AR2,P#4.0];
      L     0;
      T     DID [AR2,P#8.0]; // Ende-Kennung
//Zeiger in Kachel und AenderungsDB weiterschalten;
      L     #wSrcRecOffs;
      +AR1  ; // naechster Eintrag Aenderungs-DB
      +AR2  P#8.0; // naechster Eintrag Sendekachel
      SPA   NCPY;
NCPY: NOP   0;
      CLR   ;
      =     #bNextTile;
// Zaehler <Eintraege in Sendekachel>;
      L     #wRT;
      +     1;
      T     #wRT;
//Kachel-Bytezaehler erhoehen
      L     #wTileUsedBytes;
      L     #wTileTeleNettoLen;
      +I    ;
      T     #wTileUsedBytes;

// noch Platz? (rfe, 26.01.04)
      L     #wTileTeleNettoLen;
      +I    ;
      L     #wTileSize;
      >I    ;
      =     #bNextTile; // -> neue Kachel

//aktuellen Telegrammtyp und Zeitstempel retten;
      L     #wTeleType;
      T     #wOldTeleType;
      L     #wTimeStamp;
      T     #wOldTimeStamp;
// Zaehler <Eintraege in AenderungsDB>;
      L     #wRS;
      +     1;
      T     #wRS;
      L     #wSrcAnzDF;
      >I    ;
      SPB   XCPY; // AenderungsDB entsorgt
      UN    #bNextTile;
      SPB   LCPY; // naechsten Eintrag entsorgen
EECP: NOP   0;
//Zeiger in Aenderungs-DB merken;
      TAR1  #dArSrcDb_x;
      SPA   SEND;
XCPY: NOP   0;
//;
//AenderungsDB entsorgt (Anzahl Eintraege = 0);
//;
      LAR1  #dArSrcDb_0;
      L     0;
      T     DBW [AR1,P#0.0];
      T     #dArSrcDb_x;
//naechster DB;
      L     #wDb;
      +     1;
      T     #wDb;
      L     #wDbNo;
      +     1;
      T     #wDbNo;
      L     #wDbMaxPlus1;
      MOD   ;
      L     0;
      <>I   ;
      SPB   DBXY;
//wieder mit 1. DB beginnen
      L     1;
      T     #wDbNo;
DBXY: NOP   0;
// naechster AenderungsDB;
      SET   ;
      =     #bNextSrcDB;
SEND: NOP   0;
// Sendekachel fertig machen;
      TAR2  #dPtrUDPAct; // Kachelzeiger speichern;
      LAR2  #dPtrUDPNettoDataHeader;
//Telegrammheader aktualisieren;
      L     #wRT;
      T     DIW [AR2,P#0.0]; // Anzahl Eintraege Sendekachel;
      L     #wOldTeleType;
      T     DIW [AR2,P#2.0]; // Telegrammtyp;
      L     #wOldTimeStamp;
      T     DID [AR2,P#4.0]; // Timestamp;
      LAR2  #dPtrUDPHeader;
      L     #wTileUsedBytes;
      TAD   ;
      T     DID [AR2,P#16.0];

// rfe, 26.01.04
      SET   ;
      =     #bNewTeleHeader;

      LAR2  #dPtrUDPAct; // Kachelzeiger laden;
      UN    #bNextSrcDB;
      SPB   SNDX;
      SPA   LOP1; // naechster AenderungsDB
SNDX: NOP   0;
      SET   ;
      =     #bSendNettoData;

      L     #wPacketActWriteNdx; // aktueller Schreibindex
      T     "abvspu_DB_UDP".wPacketLastWriteNdx;
      L     1;
      +D    ;
      L     #wMaxPacketCount;
      MOD   ;
      T     #wPacketActWriteNdx; // aktueller Schreibindex (next)

      CLR   ;
      =     #bTileInUse;
      NOP   0;
// naechste Kachel;
      L     #wActPacketCountWrite;
      L     1;
      -D    ;
      T     #wActPacketCountWrite;
      L     0;
      <>D   ;
      SPB   LOP2;

      NOP   0;
//Alle Kacheln abgearbeitet;
      L     #dArSrcDb_0;
      L     0;
      <>D   ;
      SPB   ENDE;
//Anzahl Eintraege in aktuellen AenderungsDB aktualisieren;
      L     #wRS;
      +     -1;
      T     #wRS;
      AUF   DB [#wSrcDb]; // Aenderungs-DB oeffnen
      LAR1  #dArSrcDb_0;
      L     #wSrcAnzDF;
      L     #wRS;
      -I    ;
      T     DBW [AR1,P#0.0];
      L     #wSrcRecLen;
      *I    ;
      T     #wCopyAnzWords;
      L     #wRS; //Anzahl entsorgter Records
      L     #wSrcRecLen;
      *I    ;
      +     1;
      T     #wQ_Offs; //DW-Nummer des 1. zu kopierenden Records
      L     1;
      T     #wZ_Offs; //DW-Nummer des Zielbereichs
//noch nicht entsorgte Eintraege nach vorne kopieren;
      CALL "abvspu_COPY_DB" (
           ANZ_WORDS                := #wCopyAnzWords,
           Q_DBNO                   := #wSrcDb,
           Q_OFFS                   := #wQ_Offs,
           Z_DBNO                   := #wSrcDb,
           Z_OFFS                   := #wZ_Offs);

      SPA   ENDE;
NXDB: NOP   0;
//naechster DB;
      L     #wDb;
      +     1;
      T     #wDb;
      L     #wDbMaxPlus1;
      ==I   ;
      SPB   ENDE;
      L     #wDbNo;
      +     1;
      T     #wDbNo;
      L     #wDbMaxPlus1;
      MOD   ;
      L     0;
      <>I   ;
      SPB   DBXX;
//wieder mit 1. DB beginnen
      L     1;
      T     #wDbNo;
DBXX: NOP   0;
      SPA   LOP1;

ENDE: NOP   0;
      UN    #bTileInUse;
      SPB   ENDX;
// Kachel als 'sendebereit' kennzeichnen;
      L     #wPacketActWriteNdx; // aktueller Schreibindex
      T     "abvspu_DB_UDP".wPacketLastWriteNdx;
      L     1;
      +D    ;
      L     #wMaxPacketCount;
      MOD   ;
      T     #wPacketActWriteNdx; // aktueller Schreibindex (next)

      SET   ;
      =     #bSendNettoData;

ENDX: NOP   0;
      L     #wDbNo;
      T     "abvspu_DB_UDP".wActSrcDBNo;

// ##################################################################

DOXX: NOP   0;

      UN    "abvspu_DB_UDP".bSendRollbackRequest;
      SPB   QSND; // query send netto data

// ##################################################################
// handle rollback request to PC
// ##################################################################

      CALL "abvspu_UDP_NextFreeCID" ;
      T     #iActConnection;
      L     0;
      ==D   ;
      SPB   ret;

      L     "abvspu_DB_UDP".dwLastSentDataPacketId;
      TAD   ;
      T     "abvspu_DB_UDP".LifeSignTele.TeleHeader.PacketId;

//hk
      L     "abvspu_DB_UDP".dwRollbackReqReceiverId;
      TAD   ;
      T     "abvspu_DB_UDP".LifeSignTele.TeleHeader.ReceiverId;

      L     1; // packet type for rollback
      TAD   ;
      T     "abvspu_DB_UDP".LifeSignTele.TeleHeader.PacketType;

      L     4;
      TAD   ;
      T     "abvspu_DB_UDP".LifeSignTele.TeleHeader.TotalPacketLength;

      L     "abvspu_DB_UDP".wUDPHeaderSize;
      L     4; // 4 Byte Nettodaten für Rollback-ID
      +D    ;
      T     #iTmp;

      L     "abvspu_DB_UDP".dwRollbackReqPacketId;
      T     "abvspu_DB_UDP".LifeSignTele.adwData[1];

      CALL "abvspu_AGxSEND" (
           ACT                      := TRUE,
           ID                       := #iActConnection,
           LADDR                    := "abvspu_DB_UDP".wLAddr[1],
           SEND                     := "abvspu_DB_UDP".LifeSignTele,
           LEN                      := #iTmp,
           DONE                     := #snd_done,
           ERROR                    := #snd_error,
           STATUS                   := #snd_status);

      U     #snd_done;
      U     #snd_error;
      L     #snd_status;

      CLR   ;
      =     "abvspu_DB_UDP".bSendRollbackRequest;
      SPA   QSND; // query send netto data

// ##################################################################
// handle rollback request from PC
// ##################################################################
roll: NOP   0;
      CLR   ;
      =     "abvspu_DB_UDP".bRecvRollbackRequest;

      L     "abvspu_DB_UDP".wPacketLastReadNdx;
      L     "abvspu_DB_UDP".wPacketLastWriteNdx;
      >D    ;
      SPB   rb00;
      -D    ;
      L     #wMaxPacketCount;
      +D    ;
      L     "abvspu_DB_UDP".dwLastSentDataPacketId;
      >=D   ;
      SPB   rb01;
      TAK   ;
      SPA   rb01;

rb00: -D    ; // R - W
      SPA   rb01;

rb01: T     #wPacketCountRollbackMax;

// rollback ab x heißt: R soll auf Packet mit Id=x-1 zeigen
      U     "abvspu_DB_UDP".bDoRollback;
      SPBN  rb02;

// ansonsten simuliere rollback request
      L     "abvspu_DB_UDP".dwLastSentDataPacketId;
      L     "abvspu_DB_UDP".wTestRollbackCount;
      -D    ;
      L     1;
      +D    ;
      T     "abvspu_DB_UDP".dwRollbackPacketId;

rb02: CLR   ;
      =     "abvspu_DB_UDP".bDoRollback;

      L     "abvspu_DB_UDP".dwLastSentDataPacketId;
      L     "abvspu_DB_UDP".dwRollbackPacketId;

      -D    ;
      L     1;
      +D    ; // Anzahl der gewünschten Packets
      T     #iTmp;
      L     0;
      <=D   ;
      SPB   norb;

      L     #iTmp;
      L     #wPacketCountRollbackMax;
      >D    ;
      SPB   norb;

      L     "abvspu_DB_UDP".wPacketLastReadNdx;
      L     #iTmp;
      -D    ;
      L     #wMaxPacketCount;
      +D    ;
      L     #wMaxPacketCount;
      MOD   ;
      T     "abvspu_DB_UDP".wPacketLastReadNdx;

      L     "abvspu_DB_UDP".dwRollbackPacketId; // aus Telegramm
      L     "abvspu_DB_UDP".wRollbackSize; // N
      >=D   ;
      SPB   rb03;
      TAK   ;
rb03: T     "abvspu_DB_UDP".wSentPackets4Rollback; // S (max=N)
      SPA   QSND;

norb: NOP   0;
// no rollback possible (->GA)

      L     L#-1;
      T     "abvspu_DB_UDP".dwLastSentDataPacketId;
      TAD   ;
      T     "abvspu_DB_UDP".SendTeleHeader.PacketId;

      L     DW#16#FFFE;
      L     "abvspu_DB_UDP".wUDPPacketSize;
      /D    ;
      L     1;
      -D    ;
      T     "abvspu_DB_UDP".wPacketLastReadNdx;
      T     "abvspu_DB_UDP".wPacketLastWriteNdx;

      L     "abvspu_DB_UDP".wUDP_DB; // DbNo UDP-Sendepakete
      T     #wDbNo;
      AUF   DB [#wDbNo];

// clear DB191:
      L     -1;
      T     #wTmp1;
lpc:  NOP   0;
      L     #wTmp1;
      +     1;
      T     #wTmp1;
      L     DBLG;
      >=I   ;
      SPB   ftg;
      LAR1  P#DBX 0.0;
      TAK   ;
      SLD   3;
      +AR1  ;
      L     0;
      T     B [AR1,P#0.0];
      SPA   lpc;

ftg:  NOP   0;
      L     0;
      T     "abvspu_DB_UDP".dwSendBusy;

      L     "spuDB_CFG".D_52; // (HilfsDB1) DB195.DBW104
      T     #wTmp1;
      AUF   DB [#wTmp1];
      SET   ;
      =     DBX  171.0; // Generalabfrage einleiten
      =     "abvspu_DB_GLO".Tele_DT.bSend;
      CALL "abvspu_RESET_AEND_DB" ;
      SPA   ret;


// ( W + 62 - R) % 62
QSND: L     "abvspu_DB_UDP".wPacketLastWriteNdx;
      L     #wMaxPacketCount;
      +D    ;
      L     "abvspu_DB_UDP".wPacketLastReadNdx;
      -D    ;
      L     #wMaxPacketCount;
      MOD   ;
      L     0;
      <>D   ;
      SPB   sndn; // Nettodaten senden

NETWORK
TITLE =Send LifeSign

      NOP   0;

      L     "abvspu_DB_UDP".wLifeSignTimer;
      L     "abvspu_DB_GLO".Cycle1Ms;
      +D    ;
      T     "abvspu_DB_UDP".wLifeSignTimer;
      L     1000;
      <=D   ;
      SPB   ret;
      MOD   ;
      T     "abvspu_DB_UDP".wLifeSignTimer;

      U     "abvspu_DB_UDP".bLifeSignSpecial4Test;
      SPB   tst1; // Life sign Test !!

      CALL "abvspu_UDP_NextFreeCID" ;
      T     #iActConnection;
      L     0;
      ==D   ;
      SPB   ret;

      L     "abvspu_DB_UDP".dwLastSentDataPacketId;
      TAD   ;
      T     "abvspu_DB_UDP".LifeSignTele.TeleHeader.PacketId;

//hk
      L     L#-1;
//      TAD
      T     "abvspu_DB_UDP".LifeSignTele.TeleHeader.ReceiverId;

      L     2; // packet type for life sign
      TAD   ;
      T     "abvspu_DB_UDP".LifeSignTele.TeleHeader.PacketType;

      L     0;
      T     "abvspu_DB_UDP".LifeSignTele.TeleHeader.TotalPacketLength;

      L     "abvspu_DB_UDP".wUDPHeaderSize;
      T     #iTmp;

      UN    "abvspu_DB_UDP".bSendLifeSigns;
      SPB   temp;

      CALL "abvspu_AGxSEND" (
           ACT                      := TRUE,
           ID                       := #iActConnection,
           LADDR                    := "abvspu_DB_UDP".wLAddr[1],
           SEND                     := "abvspu_DB_UDP".LifeSignTele,
           LEN                      := #iTmp,
           DONE                     := #snd_done,
           ERROR                    := #snd_error,
           STATUS                   := #snd_status);

temp: NOP   0;
      SPA   ret;
NETWORK
TITLE =Send life signs for test only
//Life signs über alle verfügbaren Verbindungen senden und dabei die packet-id
//inkrementieren
tst1: NOP   0;

lp:   CALL "abvspu_UDP_NextFreeCID" ;
      T     #iActConnection;
      L     0;
      ==D   ;
      SPB   ret;


// Test: increment packet-ids
      L     "abvspu_DB_UDP".dwLastSentDataPacketId;
      L     1;
      +D    ;
      T     "abvspu_DB_UDP".dwLastSentDataPacketId;
      TAD   ;
      T     "abvspu_DB_UDP".LifeSignTele.TeleHeader.PacketId;
//

      L     "abvspu_DB_UDP".dwLastSentDataPacketId;
      TAD   ;
      T     "abvspu_DB_UDP".LifeSignTele.TeleHeader.PacketId;

      L     2; // packet type for life sign
      TAD   ;
      T     "abvspu_DB_UDP".LifeSignTele.TeleHeader.PacketType;

      L     0;
      T     "abvspu_DB_UDP".LifeSignTele.TeleHeader.TotalPacketLength;

      L     "abvspu_DB_UDP".wUDPHeaderSize;
      T     #iTmp;

      UN    "abvspu_DB_UDP".bSendLifeSigns;
      SPB   tmp2;

      CALL "abvspu_AGxSEND" (
           ACT                      := TRUE,
           ID                       := #iActConnection,
           LADDR                    := "abvspu_DB_UDP".wLAddr[1],
           SEND                     := "abvspu_DB_UDP".LifeSignTele,
           LEN                      := #iTmp,
           DONE                     := #snd_done,
           ERROR                    := #snd_error,
           STATUS                   := #snd_status);
      CALL "WAIT" (
           WT                       := 32767);
      CALL "WAIT" (
           WT                       := 32767);
      CALL "WAIT" (
           WT                       := 32767);

      SPA   lp; //nur für Test

tmp2: NOP   0;
      SPA   ret;



NETWORK
TITLE =UDP-Pakete senden

sndn: NOP   0;

// Max. Anzahl zu sendender Packets ermitteln
// (W + 62 - R) % 62
      L     "abvspu_DB_UDP".wPacketLastWriteNdx;
      L     #wMaxPacketCount;
      +D    ;
      L     "abvspu_DB_UDP".wPacketLastReadNdx;
      -D    ;
      L     #wMaxPacketCount;
      MOD   ;
      T     #wActPacketCountRead; // = max. Anzahl

      L     "abvspu_DB_UDP".wPacketLastReadNdx;
      L     1;
      +D    ;
      L     #wMaxPacketCount;
      MOD   ;
      T     #wPacketActReadNdx; // aktueller Leseindex für Senden

// Unabhängig von Rollback: ALLE Packets senden
      L     #wActPacketCountRead;
      L     0;
      ==D   ;
      SPB   ret; // keine Packets

lpsn: NOP   0; // loop for send
      L     #wPacketActReadNdx;
      L     "abvspu_DB_UDP".wUDPPacketSize;
      *D    ;
      SLD   3;
      LAR2  ;
      AUF   DI [#wUDP_DataDB];

      L     W#16#1002;
      T     LW     0;
      L     "abvspu_DB_UDP".wUDPPacketSize;
      T     LW     2;
      L     #wUDP_DataDB;
      T     LW     4;
      L     P#DBX 0.0; // == dw#16#84000000
      TAR2  ;
      +D    ;
      LAR2  ;
      T     LD     6;

      AUF   DB [#wUDP_DataDB];
      L     D [AR2,P#4.0]; // == m_lPacketId
      TAD   ;
      T     #dwTmpPacketId;
      L     D [AR2,P#16.0]; // == m_lTotalPacketLength
      TAD   ;
      L     "abvspu_DB_UDP".wUDPHeaderSize;
      +D    ;
      T     #iTmp;

      CALL "abvspu_UDP_NextFreeCID" ;
      T     #iActConnection;
      L     0;
      ==D   ;
      SPB   ret;


//hallo provoziere, dass PLC mit viel zu kleinen (20 < rollbacksize)
// packet ids sendet:

//      U     DB190.DBX  400.0
//      SPBN  hlo
//      R     DB190.DBX  400.0
//      AUF   DB [#wUDP_DataDB]
//      L     D [AR2,P#4.0]
//      TAD
//      L     20
//      -D
//      TAD
//      T     D [AR2,P#4.0]



      CALL "abvspu_AGxSEND" (
           ACT                      := FALSE,
           ID                       := #iActConnection,
           LADDR                    := "abvspu_DB_UDP".wLAddr[1],
           SEND                     := #anyPtrSend,
           LEN                      := #iTmp,
           DONE                     := #snd_done,
           ERROR                    := #snd_error,
           STATUS                   := #snd_status);

      L     #iTmp;
      L     "abvspu_DB_UDP".wLastSentPacketLength;
      >=D   ;
      SPB   cont;

      CALL "WAIT" (
           WT                       := 10000);

cont: NOP   0;
      L     #iTmp;
      T     "abvspu_DB_UDP".wLastSentPacketLength;


s000: CALL "abvspu_AGxSEND" (
           ACT                      := TRUE,
           ID                       := #iActConnection,
           LADDR                    := "abvspu_DB_UDP".wLAddr[1],
           SEND                     := #anyPtrSend,
           LEN                      := #iTmp,
           DONE                     := #snd_done,
           ERROR                    := #snd_error,
           STATUS                   := #snd_status);

      UN    "abvspu_DB_UDP".bIs400;
      UN    #snd_done;
      UN    #snd_error;
      SPB   s000;

////////////////////////////////////////////////////////////
      TAR2  #dwTmpAR2;

      LAR2  "abvspu_DB_UDP".dPtrLastSentDataLength;
      L     #iActConnection;
      L     "abvspu_DB_UDP".wFirstConnection;
      -D    ;
      SLD   4; //*2 (WORD), *8 (Pointer)
      +AR2  ;
      L     LW     2; // Längenangabe aus anyPtrSend
      T     W [AR2,P#0.0];

      LAR2  "abvspu_DB_UDP".dPtrLastDataPtr;
      L     #iActConnection;
      L     "abvspu_DB_UDP".wFirstConnection;
      -D    ;
      SLD   5; //*4 (DWORD), *8 (Pointer)
      +AR2  ;
      L     LD     6; // Ber.übergr.Zeiger aus anyPtrSend
      T     D [AR2,P#0.0];

      LAR2  #dwTmpAR2;
////////////////////////////////////////////////////

      L     #iActConnection;
      L     "abvspu_DB_UDP".wFirstConnection;
      -D    ;
      L     1;
      SLD   ;

      L     "abvspu_DB_UDP".dwSendBusy;
      OD    ;
      T     "abvspu_DB_UDP".dwSendBusy;


// later: send twice on 2 LAddr, hallo

      L     #dwTmpPacketId;
      L     W#16#FFF;
      UD    ; // 12 Bit reichen
      L     #iActConnection;
      SLD   12;
      OD    ;
      T     #iTmp;

      UN    #snd_error;
      SPB   e005;

      L     #dwTmpPacketId;
      T     "abvspu_DB_UDP".dwErrorPacketId;

e005: NOP   0;

      UN    #bWrite2Logfile;
      SPB   NLOG;

// write to logfile
      TAR2  #dwTmpAR2;
      LAR2  "abvspu_DB_UDP".ptrUDPLog;
      L     "abvspu_DB_UDP".wUDPLogDBNo;
      T     #wTmpUDPLogDBNo;
      AUF   DB [#wTmpUDPLogDBNo];
      L     #iTmp;
      T     W [AR2,P#0.0];
      L     #snd_status;
      T     W [AR2,P#2.0];
      TAR2  ;
      L     P#4.0;
      +D    ;
      L     P#DBX 2047.7;
      UD    ;
      T     "abvspu_DB_UDP".ptrUDPLog;

      NOP   0;
      L     "abvspu_DB_UDP".wSentPackets4Rollback;
      L     "abvspu_DB_UDP".wRollbackSize;
      >=D   ;
      SPB   tmp;
      TAK   ;
      L     1;
      +D    ;
      T     "abvspu_DB_UDP".wSentPackets4Rollback;

tmp:  LAR2  #dwTmpAR2;
// ende: write to logfile

NLOG: NOP   0;
      L     DID [AR2,P#4.0];
      TAD   ;
      T     "abvspu_DB_UDP".dwLastSentDataPacketId;

      L     #wPacketActReadNdx; // aktueller Leseindex für Senden
      T     "abvspu_DB_UDP".wPacketLastReadNdx;
      L     1;
      +D    ;

//hk
      L     #wMaxPacketCount;
      MOD   ;

      T     #wPacketActReadNdx;

      L     #wActPacketCountRead;
      L     1;
      -D    ;
      T     #wActPacketCountRead;
      L     0;
      ==D   ;
      SPB   ret; // alle Packets versendet
      SPA   lpsn;
NETWORK
TITLE =Ende

ret:  BE    ;

END_FUNCTION

